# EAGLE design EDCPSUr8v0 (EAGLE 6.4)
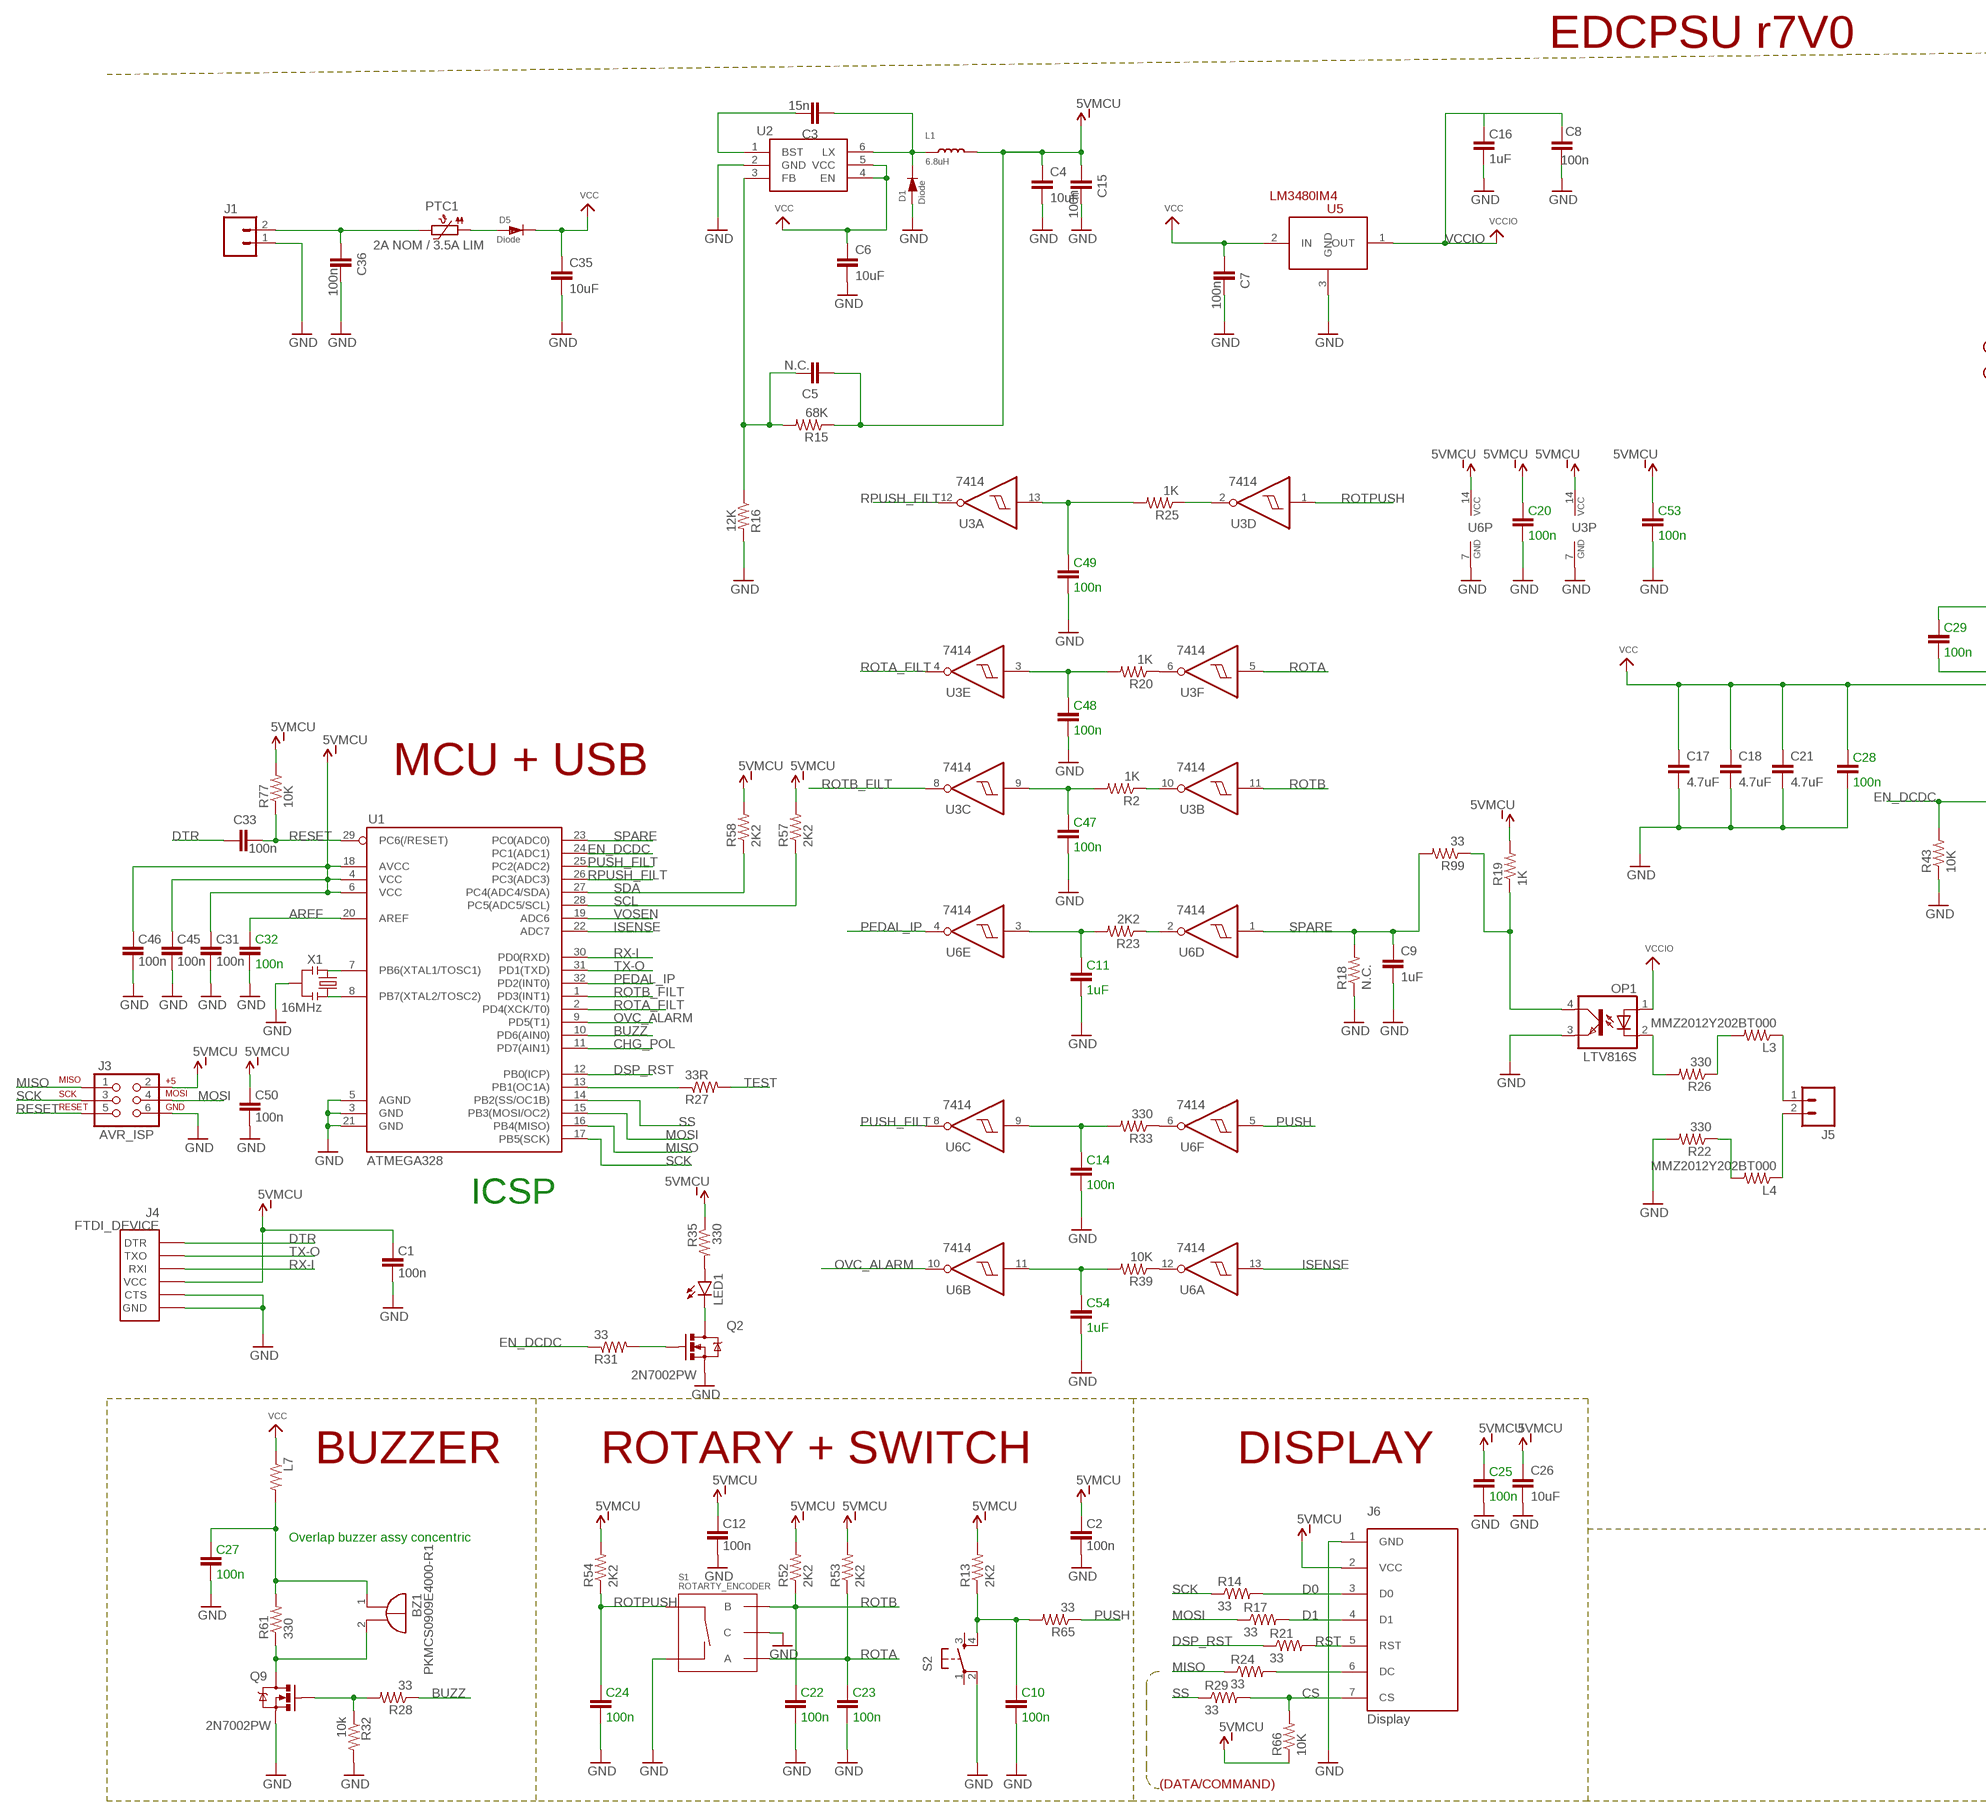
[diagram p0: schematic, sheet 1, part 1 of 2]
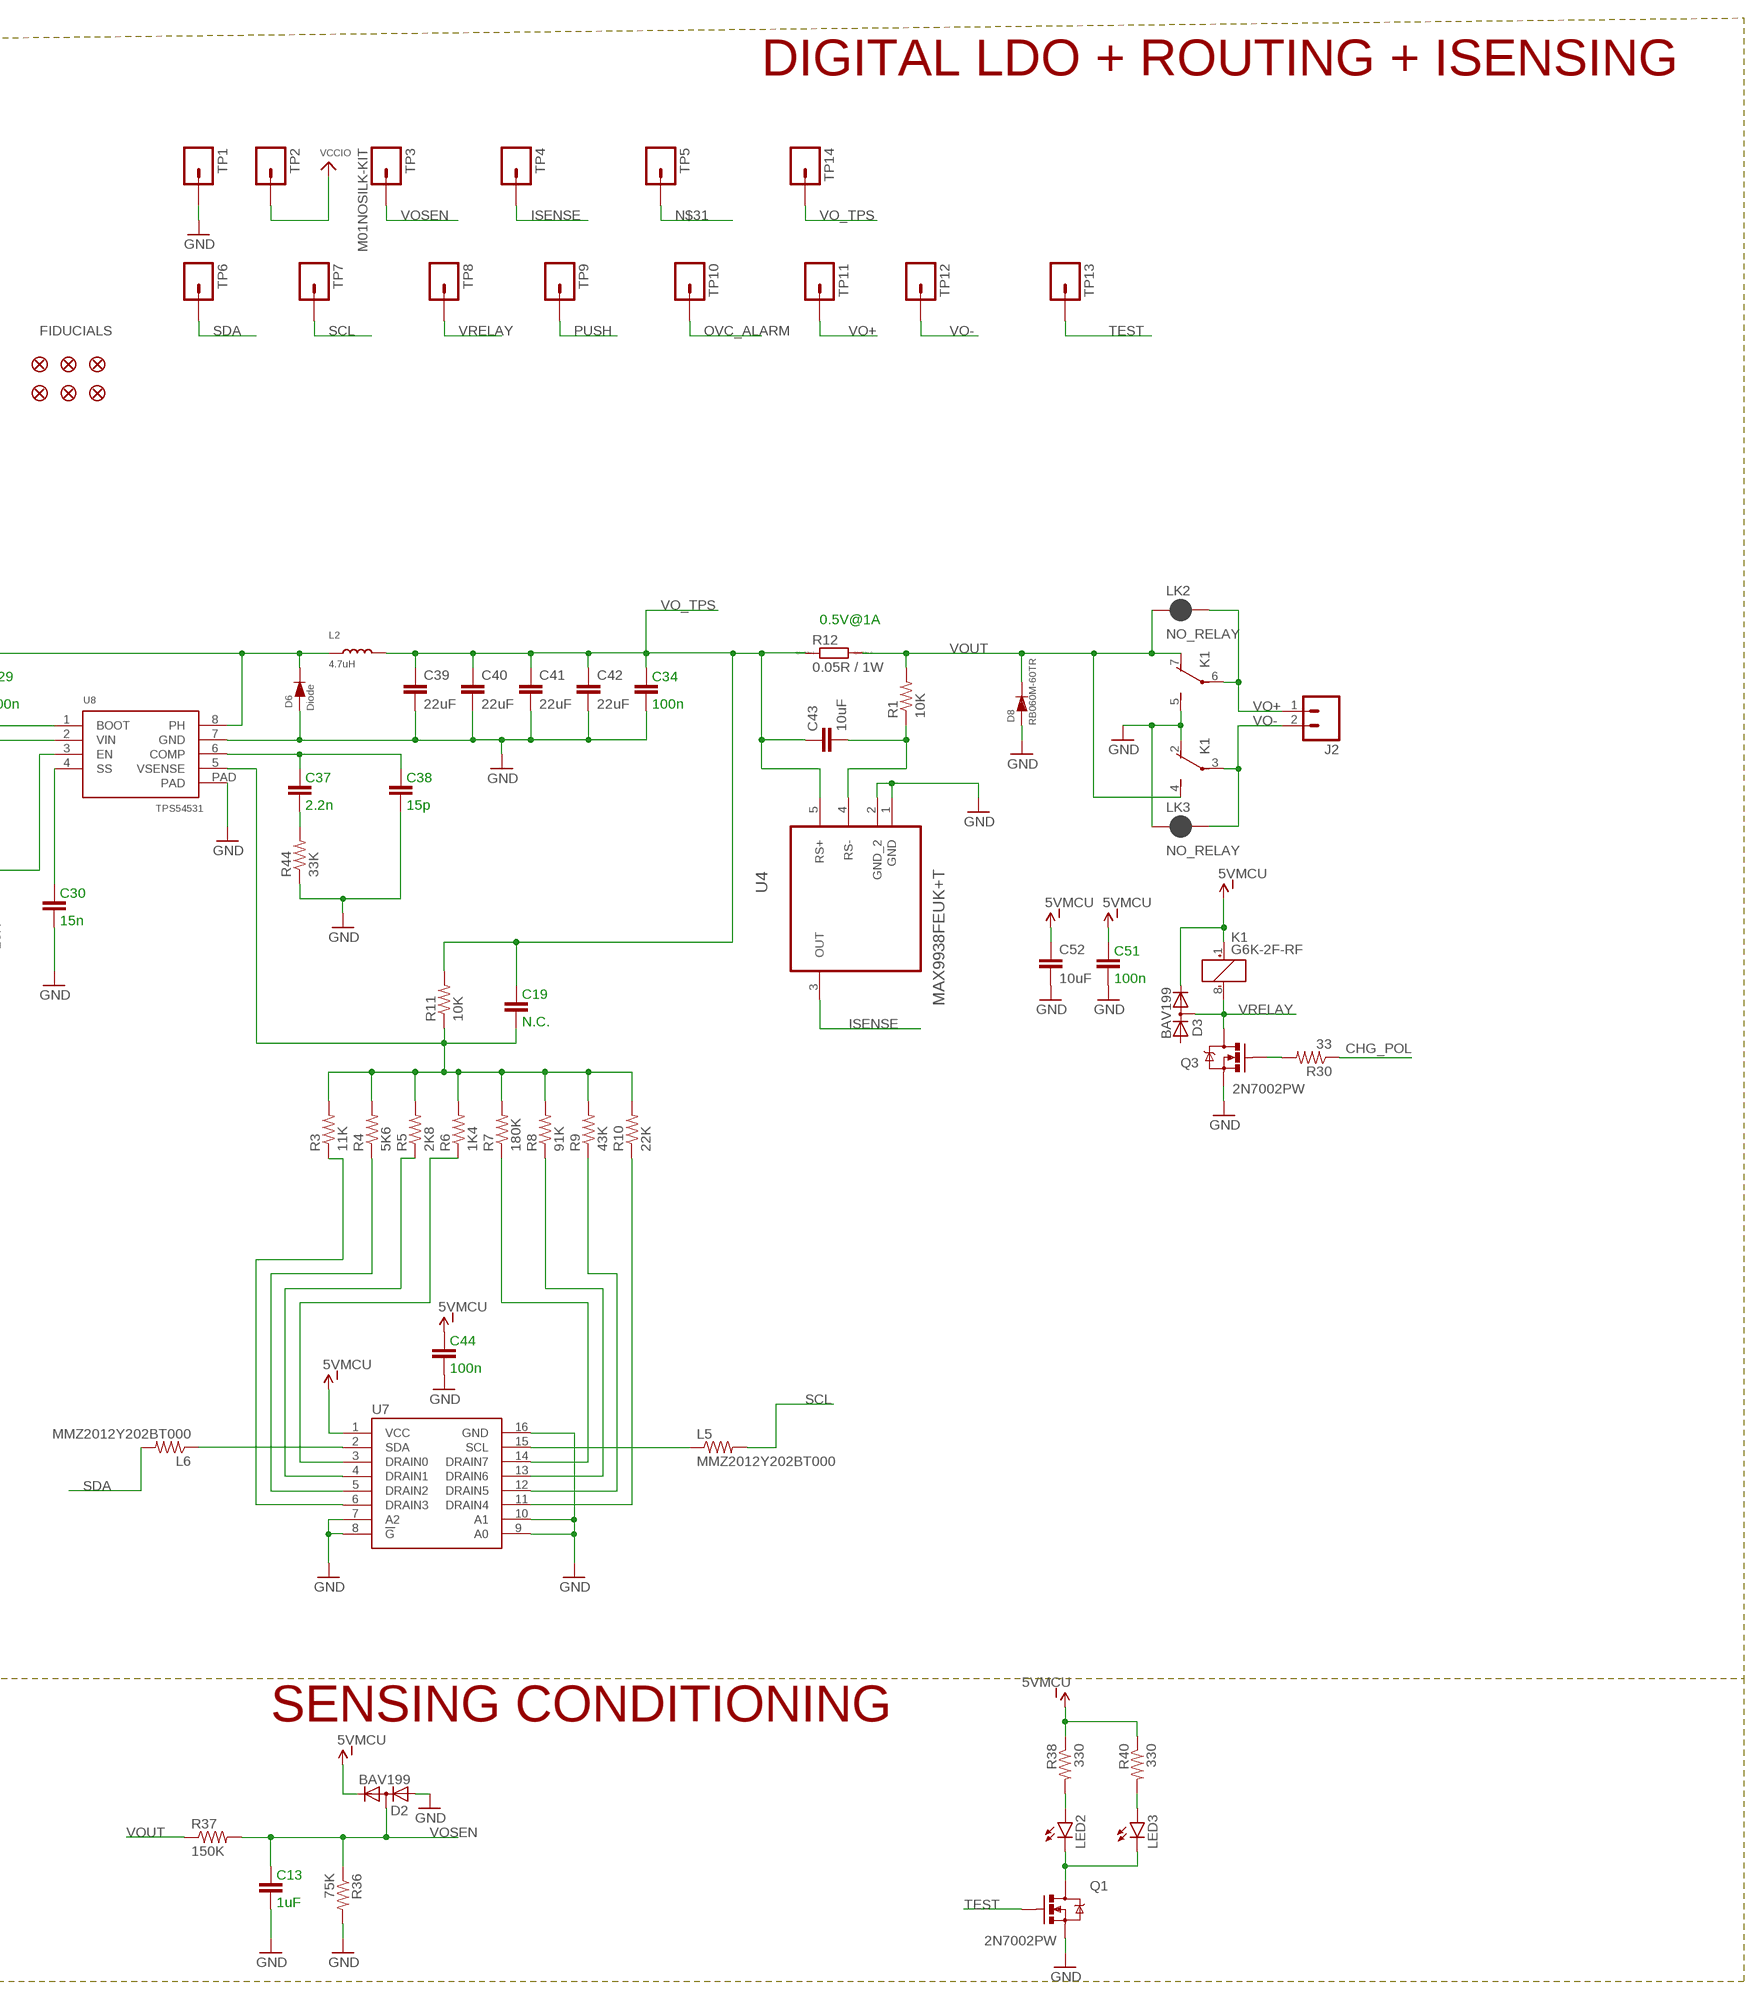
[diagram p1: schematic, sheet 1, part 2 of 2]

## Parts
BZ1  PKMCS0909E4000-R1  [PKMCS0909]
C1  100n  CAP0805  [0805]
C2  100n  CAP0805  [0805]
C3  15n  CAP0805  [0805]
C4  10uF  CAP1206  [1206]
C5  N.C.  CAP0805  [0805]
C6  10uF  CAP1206  [1206]
C7  100n  CAP0805  [0805]
C8  100n  CAP0805  [0805]
C9  1uF  CAP1206  [1206]
C10  100n  CAP0805  [0805]
C11  1uF  CAP0805  [0805]
C12  100n  CAP0805  [0805]
C13  1uF  CAP0805  [0805]
C14  100n  CAP0805  [0805]
C15  100n  CAP0805  [0805]
C16  1uF  CAP0805  [0805]
C17  4.7uF  CAP1210  [1210]
C18  4.7uF  CAP1210  [1210]
C19  N.C.  CAP0805  [0805]
C20  100n  CAP0805  [0805]
C21  4.7uF  CAP1210  [1210]
C22  100n  CAP0805  [0805]
C23  100n  CAP0805  [0805]
C24  100n  CAP0805  [0805]
C25  100n  CAP0805  [0805]
C26  10uF  CAP1206  [1206]
C27  100n  CAP0805  [0805]
C28  100n  CAP0805  [0805]
C29  100n  CAP0805  [0805]
C30  15n  CAP0805  [0805]
C31  100n  CAP0805  [0805]
C32  100n  CAP0805  [0805]
C33  100n  CAP0805  [0805]
C34  100n  CAP0805  [0805]
C35  10uF  CAP1206  [1206]
C36  100n  CAP0805  [0805]
C37  2.2n  CAP0805  [0805]
C38  15p  CAP0805  [0805]
C39  22uF  CAP1210  [1210]
C40  22uF  CAP1210  [1210]
C41  22uF  CAP1210  [1210]
C42  22uF  CAP1210  [1210]
C43  10uF  CAP1206  [1206]
C44  100n  CAP0805  [0805]
C45  100n  CAP0805  [0805]
C46  100n  CAP0805  [0805]
C47  100n  CAP0805  [0805]
C48  100n  CAP0805  [0805]
C49  100n  CAP0805  [0805]
C50  100n  CAP0805  [0805]
C51  100n  CAP0805  [0805]
C52  10uF  CAP1206  [1206]
C53  100n  CAP0805  [0805]
C54  1uF  CAP0805  [0805]
D1  Diode  DSOD123  [SOD123]
D2  BAV199  [SOT23]
D3  BAV199  [SOT23]
D5  Diode  DSMC  [DO-214AB]
D6  Diode  DSMC  [DO-214AB]
D8  RB060M-60TR  DSMA  [SMADIODE]
FID1  FIDUCIAL1X2  [FIDUCIAL-1X2]
FID2  FIDUCIAL1X2  [FIDUCIAL-1X2]
FID3  FIDUCIAL1X2  [FIDUCIAL-1X2]
FID4  FIDUCIAL1X2  [FIDUCIAL-1X2]
FID5  FIDUCIAL1X2  [FIDUCIAL-1X2]
FID6  FIDUCIAL1X2  [FIDUCIAL-1X2]
J1  M02LOCK_LONGPADS  [1X02_LOCK_LONGPADS]
J2  M02LOCK_LONGPADS  [1X02_LOCK_LONGPADS]
J3  AVR_ISP  AVR_SPI_PRG_62X3_LOCK  [2X3_LOCK]
J4  FTDI_DEVICE  [FTDI_DEVICE_SIDE]
J5  M02LOCK_LONGPADS  [1X02_LOCK_LONGPADS]
J6  Display  OLED_LCD  [OLED_LCD]
K1  G6K-2F-RF  [G6K-RF]
L1  6.8uH  L4018  [NR4018T100M]
L2  4.7uH  L74437368047  [WE-LHMI]
L3  MMZ2012Y202BT000  RESISTOR0805-RES  [0805]
L4  MMZ2012Y202BT000  RESISTOR0805-RES  [0805]
L5  MMZ2012Y202BT000  RESISTOR0805-RES  [0805]
L6  MMZ2012Y202BT000  RESISTOR0805-RES  [0805]
L7  MMZ2012Y202BT000  RESISTOR0805-RES  [0805]
LED1  LED3MM  [LED3MM]
LED2  LED5MM  [LED5MM]
LED3  LED5MM  [LED5MM]
LK2  NO_RELAY  JUMPER-PAD-2-NC_BY_PASTE  [PAD-JUMPER-2-NC_BY_PASTE_YES_SILK]
LK3  NO_RELAY  JUMPER-PAD-2-NC_BY_PASTE  [PAD-JUMPER-2-NC_BY_PASTE_YES_SILK]
OP1  LTV816S  [SMD4]
PTC1  2A NOM / 3.5A LIM  PTC-  [1812L]
Q1  2N7002PW  MOSFET-NCHANNEL2N7002PW  [SOT323]
Q2  2N7002PW  MOSFET-NCHANNEL2N7002PW  [SOT323]
Q3  2N7002PW  MOSFET-NCHANNEL2N7002PW  [SOT323]
Q9  2N7002PW  MOSFET-NCHANNEL2N7002PW  [SOT323]
R1  10K  RESISTOR0805-RES  [0805]
R2  1K  RESISTOR0805-RES  [0805]
R3  11K  RESISTOR0805-RES  [0805]
R4  5K6  RESISTOR0805-RES  [0805]
R5  2K8  RESISTOR0805-RES  [0805]
R6  1K4  RESISTOR0805-RES  [0805]
R7  180K  RESISTOR0805-RES  [0805]
R8  91K  RESISTOR0805-RES  [0805]
R9  43K  RESISTOR0805-RES  [0805]
R10  22K  RESISTOR0805-RES  [0805]
R11  10K  RESISTOR0805-RES  [0805]
R12  0.05R / 1W  RR2512  [R2512]
R13  2K2  RESISTOR0805-RES  [0805]
R14  33  RESISTOR0805-RES  [0805]
R15  68K  RESISTOR0805-RES  [0805]
R16  12K  RESISTOR0805-RES  [0805]
R17  33  RESISTOR0805-RES  [0805]
R18  N.C.  RESISTOR0805-RES  [0805]
R19  1K  RESISTOR0805-RES  [0805]
R20  1K  RESISTOR0805-RES  [0805]
R21  33  RESISTOR0805-RES  [0805]
R22  330  RESISTOR1206  [1206]
R23  2K2  RESISTOR0805-RES  [0805]
R24  33  RESISTOR0805-RES  [0805]
R25  1K  RESISTOR0805-RES  [0805]
R26  330  RESISTOR1206  [1206]
R27  33R  RESISTOR0805-RES  [0805]
R28  33  RESISTOR0805-RES  [0805]
R29  33  RESISTOR0805-RES  [0805]
R30  33  RESISTOR0805-RES  [0805]
R31  33  RESISTOR0805-RES  [0805]
R32  10k  RESISTOR0805-RES  [0805]
R33  330  RESISTOR0805-RES  [0805]
R35  330  RESISTOR0805-RES  [0805]
R36  75K  RESISTOR0805-RES  [0805]
R37  150K  RESISTOR0805-RES  [0805]
R38  330  RESISTOR0805-RES  [0805]
R39  10K  RESISTOR0805-RES  [0805]
R40  330  RESISTOR0805-RES  [0805]
R43  10K  RESISTOR0805-RES  [0805]
R44  33K  RESISTOR0805-RES  [0805]
R52  2K2  RESISTOR0805-RES  [0805]
R53  2K2  RESISTOR0805-RES  [0805]
R54  2K2  RESISTOR0805-RES  [0805]
R57  2K2  RESISTOR0805-RES  [0805]
R58  2K2  RESISTOR0805-RES  [0805]
R61  330  RESISTOR0805-RES  [0805]
R65  33  RESISTOR0805-RES  [0805]
R66  10K  RESISTOR0805-RES  [0805]
R77  10K  RESISTOR0805-RES  [0805]
R99  33  RESISTOR0805-RES  [0805]
S1  ROTARTY_ENCODER  [ROTARY_ENC_PLAIN]
S2  TAC_SWITCH_KSC931G-SMD  [TAC_SW_SMD_KSC931G]
TP1  M01POGOPIN_HOLE_LARGE  [1X01_POGOPIN_HOLE_LARGE]
TP2  M01POGOPIN_HOLE_LARGE  [1X01_POGOPIN_HOLE_LARGE]
TP3  M01NOSILK-KIT  [1X01NS-KIT]
TP4  M01POGOPIN_HOLE_LARGE  [1X01_POGOPIN_HOLE_LARGE]
TP5  M01POGOPIN_HOLE_LARGE  [1X01_POGOPIN_HOLE_LARGE]
TP6  M01POGOPIN_HOLE_LARGE  [1X01_POGOPIN_HOLE_LARGE]
TP7  M01POGOPIN_HOLE_LARGE  [1X01_POGOPIN_HOLE_LARGE]
TP8  M01POGOPIN_HOLE_LARGE  [1X01_POGOPIN_HOLE_LARGE]
TP9  M01POGOPIN_HOLE_LARGE  [1X01_POGOPIN_HOLE_LARGE]
TP10  M01POGOPIN_HOLE_LARGE  [1X01_POGOPIN_HOLE_LARGE]
TP11  M01POGOPIN_HOLE_LARGE  [1X01_POGOPIN_HOLE_LARGE]
TP12  M01POGOPIN_HOLE_LARGE  [1X01_POGOPIN_HOLE_LARGE]
TP13  M01POGOPIN_HOLE_LARGE  [1X01_POGOPIN_HOLE_LARGE]
TP14  M01POGOPIN_HOLE_LARGE  [1X01_POGOPIN_HOLE_LARGE]
U1  ATMEGA328  ATMEGA168  [TQFP32-08]
U2  BD9G101G  [SSOP6]
U3  7414  [TSSOP14]
U4  MAX9938FEUK+T  [SOT95P280X145-5N]
U5  LM3480IM4  [SOT23-3]
U6  7414  [TSSOP14]
U7  TPIC2810D  [SO16]
U8  TPS54531  TPS5431DDAR  [SOIC8]
X1  16MHz  RESONATORSMD  [RESONATOR-SMD]

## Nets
AREF: C32.2 U1.20(AREF)
BUZZ: R28.1 U1.10(PD6(AIN0))
CHG_POL: R30.1 U1.11(PD7(AIN1))
CS: J6.7(CS) R29.2 R66.2
D0: J6.3(D0) R14.2
D1: J6.4(D1) R17.2
DSP_RST: R21.1 U1.12(PB0(ICP))
DTR: C33.2 J4.P$1(DTR)
EN_DCDC: R31.1 R43.2 U1.24(PC1(ADC1)) U8.3(EN)
GND: C1.1 C2.1 C4.2 C6.2 C7.1 C8.1 C9.2 C10.1 C11.1 C12.1 C13.1 C14.1 C15.1 C16.1 C17.2 C18.2 C20.1 C21.2 C22.1 C23.1 C24.1 C25.1 C26.2 C27.1 C28.1 C30.1 C31.1 C32.1 C34.1 C35.2 C36.1 C38.1 C39.2 C40.2 C41.2 C42.2 C44.1 C45.1 C46.1 C47.1 C48.1 C49.1 C50.1 C51.1 C52.2 C53.1 C54.1 D1.+(A) D2.1(A) D6.1(A) D8.A J1.1 J3.6 J4.P$5(CTS) J4.P$6(GND) J6.1(GND) K1.2(A:O) K1.5(B:S) LK3.1 OP1.3(EMIT) Q1.2(S) Q2.2(S) Q3.2(S) Q9.2(S) R16.2 R18.1 R22.2 R32.2 R36.2 R43.1 R44.1 S1.C S1.SW- S2.2 TP1.1 U1.3(GND) U1.5(AGND) U1.21(GND) U2.2(GND) U3.7(P:GND) U4.1(GND) U4.2(GND_2) U5.3(GND) U6.7(P:GND) U7.7(A2) U7.8(!G) U7.9(A0) U7.10(A1) U7.16(GND) U8.7(GND) U8.PAD X1.2
ISENSE: TP4.1 U1.22(ADC7) U4.3(OUT) U6.13(A:I)
MISO: J3.1 R24.1 U1.16(PB4(MISO))
MOSI: J3.4 R17.1 U1.15(PB3(MOSI/OC2))
N$1: R3.1 U7.6(DRAIN3)
N$2: R4.1 U7.5(DRAIN2)
N$3: R5.1 U7.4(DRAIN1)
N$4: R6.1 U7.3(DRAIN0)
N$5: R7.1 U7.14(DRAIN7)
N$6: J6.6(DC) R24.2
N$7: R8.1 U7.13(DRAIN6)
N$8: R9.1 U7.12(DRAIN5)
N$9: R10.1 U7.11(DRAIN4)
N$10: C43.2 R1.1 U4.4(RS-)
N$11: LED1.A R35.2
N$12: LED1.K(C) Q2.3(D)
N$13: R33.1 U6.6(F:O)
N$14: D5.1(A) PTC1.1
N$15: R39.1 U6.12(A:O)
N$16: C3.1 U2.1(BST)
N$17: C10.2 R13.1 R65.2 S2.4
N$18: C47.2 R2.2 U3.9(C:I)
N$19: C3.2 D1.-(K) L1.1 U2.6(LX)
N$20: Q9.1(G) R28.2 R32.1
N$21: Q2.1(G) R31.2
N$22: R2.1 U3.10(B:O)
N$23: R20.1 U3.6(F:O)
N$24: U1.8(PB7(XTAL2/TOSC2)) X1.1
N$25: R25.1 U3.2(D:O)
N$26: C49.2 R25.2 U3.13(A:I)
N$27: C5.1 R15.2 R16.1 U2.3(FB)
N$28: C48.2 R20.2 U3.3(E:I)
N$29: C11.2 R23.2 U6.3(E:I)
N$30: R27.1 U1.13(PB1(OC1A))
N$31: OP1.4(COL) R19.1 R99.1 TP5.1
N$32: BZ1.1(+) C27.2 L7.2 R61.2
N$33: C36.2 J1.2 PTC1.2
N$34: R23.1 U6.2(D:O)
N$36: U1.7(PB6(XTAL1/TOSC1)) X1.3
N$37: C14.2 R33.2 U6.9(C:I)
N$38: LED2.A R38.2
N$39: C54.2 R39.2 U6.11(B:I)
N$40: L6.1 U7.2(SDA)
N$41: OP1.2(C) R26.2
N$42: Q3.1(G) R30.2
N$43: L3.2 R26.1
N$44: C30.2 U8.4(SS)
N$46: L4.2 R22.1
N$47: C29.1 U8.1(BOOT)
N$48: C19.1 R3.2 R4.2 R5.2 R6.2 R7.2 R8.2 R9.2 R10.2 R11.1 U8.5(VSENSE)
N$49: LED3.A R40.2
N$51: C29.2 D6.2(K) L2.1 U8.8(PH)
N$52: C37.2 C38.2 U8.6(COMP)
N$53: C37.1 R44.2
N$54: L5.1 U7.15(SCL)
N$55: J5.1 L3.1
N$56: J5.2 L4.1
N$57: LED2.K(C) LED3.K(C) Q1.3(D)
N$64: BZ1.2(-) Q9.3(D) R61.1
OVC_ALARM: TP10.1 U1.9(PD5(T1)) U6.10(B:O)
PEDAL_IP: U1.32(PD2(INT0)) U6.4(E:O)
PUSH: R65.1 TP9.1 U6.5(F:I)
PUSH_FILT: U1.25(PC2(ADC2)) U6.8(C:O)
RESET: C33.1 J3.5 R77.1 U1.29(PC6(/RESET))
ROTA: C23.2 R53.1 S1.A U3.5(F:I)
ROTA_FILT: U1.2(PD4(XCK/T0)) U3.4(E:O)
ROTB: C22.2 R52.1 S1.B U3.11(B:I)
ROTB_FILT: U1.1(PD3(INT1)) U3.8(C:O)
ROTPUSH: C24.2 R54.1 S1.SW+ U3.1(D:I)
RPUSH_FILT: U1.26(PC3(ADC3)) U3.12(A:O)
RST: J6.5(RST) R21.2
RX-I: J4.P$3(RXI) U1.30(PD0(RXD))
SCK: J3.3 R14.1 U1.17(PB5(SCK))
SCL: L5.2 R57.1 TP7.1 U1.28(PC5(ADC5/SCL))
SDA: L6.2 R58.1 TP6.1 U1.27(PC4(ADC4/SDA))
SPARE: C9.1 R18.2 R99.2 U1.23(PC0(ADC0)) U6.1(D:I)
SS: R29.1 U1.14(PB2(SS/OC1B))
TEST: Q1.1(G) R27.2 TP13.1
TX-O: J4.P$2(TXO) U1.31(PD1(TXD))
VCC: C6.1 C7.2 C17.1 C18.1 C21.1 C28.2 C35.1 D5.2(K) L7.1 U2.4(EN) U2.5(VCC) U5.2(IN) U8.2(VIN)
VCC-ISO: C1.2 C2.2 C4.1 C5.2 C12.2 C15.2 C20.2 C25.2 C26.1 C31.2 C44.2 C45.2 C46.2 C50.2 C51.2 C52.1 C53.2 D2.2(C) D3.2(C) J3.2 J4.P$4(VCC) J6.2(VCC) K1.1(1:+) L1.2 R13.2 R15.1 R19.2 R35.1 R38.1 R40.1 R52.2 R53.2 R54.2 R57.2 R58.2 R66.1 R77.2 U1.4(VCC) U1.6(VCC) U1.18(AVCC) U3.14(P:VCC) U6.14(P:VCC) U7.1(VCC) ; supply symbol labelled 5VMCU
VCCIO: C8.2 C16.2 OP1.1(A) TP2.1 U5.1(OUT)
VO+: J2.1 K1.6(B:P) LK2.2 TP11.1
VO-: J2.2 K1.3(A:P) LK3.2 TP12.1
VO_TPS: C19.2 C34.2 C39.1 C40.1 C41.1 C42.1 C43.1 L2.2 R11.2 R12.1 TP14.1 U4.5(RS+)
VOSEN: C13.2 D2.3(AC) R36.1 R37.2 TP3.1 U1.19(ADC6)
VOUT: D8.C(K) K1.4(A:S) K1.7(B:O) LK2.1 R1.2 R12.2 R37.1
VRELAY: D3.3(AC) K1.8(1:-) Q3.3(D) TP8.1
Unconnected: D3.1(A) K1.A(S1:SH) K1.B(S2:SH) S2.1 S2.3

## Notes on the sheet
- EDCPSU r7V0
- DIGITAL LDO + ROUTING + ISENSING
- FIDUCIALS
- 0.5V@1A
- MCU + USB
- ICSP
- BUZZER | ROTARY + SWITCH | DISPLAY
- Overlap buzzer assy concentric
- SENSING CONDITIONING
- (DATA/COMMAND)

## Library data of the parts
BZ1 = buzzer:PKMCS0909E4000-R1: PKMCS0909E4000-R1
C1-C3 C5 C7 C8 C10-C16 C19 C20 C22-C25 C27-C34 C36-C38 C44-C51 C53 C54 = SparkFun:CAP: Capacitor
C4 C6 C9 C17 C18 C21 C26 C35 C39-C43 C52 = SparkFun-Passives:CAP: Capacitor
D1 D5 D6 D8 = EDCPSU - Rev3:D*
D2 D3 = diode:BAV199: DIODE low-leakage double diode
FID1-FID6 = SparkFun-Aesthetics:FIDUCIAL: Fiducial Alignment Points
J1 J2 J5 = SparkFun-Connectors:M02: Standard 2-pin 0.1" header. Use with
J3 = SparkFun-Connectors:AVR_SPI_PRG_6: AVR ISP 6 Pin This is the reduced ISP connector for AVR programming. Common on Arduino. This footprint will take up less PCB space and can be used with a 10-pin to 6-pin adapter such as SKU: BOB-08508 **Special note about "TEST_POINT" package. The stop mask is on the top side, so if you want your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
J4 = SparkFun-Connectors:FTDI_DEVICE: Connector which mates to FTDI basic or FTDI cable.
J6 = EDCPSU:OLED_LCD
K1 = relay:G6K*-2F-RF: OMRON High Frequency Relay G6K-RF Compact High Frequency Relays with 2 Form C (DPDT) Contacts Handles 1 A, 30 VDC discrete load and 1 W at 1 GHz high frequency load D20G6KRF0602.pdf; MF: OMRON COMPONENTS USA; MPN: G6K-2F-RF-DC12; OC_FARNELL: 1448181; OC_NEWARK: 73C8948
L1 L2 = EDCPSU - Rev3:L*
L3-L7 R1-R11 R13-R21 R23-R25 R27-R33 R35-R40 R43 R44 R52-R54 R57 R58 R61 R65 R66 R77 R99 = SparkFun:RESISTOR: Resistor
LED1-LED3 = SparkFun-LED:LED: LEDs
LK2 LK3 = SparkFun-Passives:JUMPER-PAD-2-NC_BY_PASTE
OP1 = optocoupler:LTV816: OPTO COUPLER Source: LITEON, LTV816.pdf; OC_FARNELL: unknown; OC_NEWARK: unknown
PTC1 = EDCPSU:PTC-: Positive Temperature Coefficient Resistor (PTC)
Q1-Q3 Q9 = SparkFun-DiscreteSemi:MOSFET-NCHANNEL: Common NMOSFET Parts MFG P/NStore IDProd ID FDD8780TRANS-09984 SI7820DNTRANS-11055 FDS6630AIC-08089 2N7002PWTRANS-11151 FQP30N06L COM-10213TRANS-10060 BSS123LT1GTRANS-08345 BSS138TRANS-00830 BS170 2N7000; PROD_ID: TRANS-11151
R12 = eagle-ltspice:R: RESISTOR, European symbol; SPICEMODEL: NONE; SPICEPREFIX: R
R22 R26 = SparkFun-Passives:RESISTOR: Resistor
S1 = SparkFun-Electromechanical:ROTARTY_ENCODER: Simple no LED rotary encoder Example: COM-09117
S2 = EDCPSU - Rev2:TAC_SWITCH: Momentary Switch Button commonly used for reset or general input. Spark Fun Electronics SKU : COM-00097 SMT- SWCH-08247
TP1-TP14 = SparkFun-Connectors:M01: Header 1
U1 = SparkFun:ATMEGA168
U2 = EDCPSU - Rev3:BD9G101G: BD9G101G - Simple Step-down Switching Regulators with Built-in Power MOSFET
U3 U6 = 74xx-eu:74*14: Hex schmitt trigger INVERTER
U4 = MAX9938:MAX9938FEUK+T; DESCRIPTION: Precision Current-Sense Amplifier; MPN: MAX9938FEUK+T; OC_FARNELL: -; OC_NEWARK: 01N6733; PACKAGE: SOT-23-5; SUPPLIER: Maxim
U5 = SparkFun-PowerIC:LM3480IM4: Small package linear regulator
U7 = EDCPSU - Rev2:TPIC2810D
U8 = EDCPSU - Rev3:TPS5431DDAR: Source : http://www.ti.com/lit/ds/symlink/tps54531.pdf
X1 = SparkFun:RESONATOR: Resonator Small SMD resonator. This is the itty bitty 10/20MHz resonators with built in caps. CSTCE10M0G55 and CSTCE20M0V53. Footprint has been reviewed closely but hasn't been tested yet.

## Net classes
1 vcc: width 0.254 mm

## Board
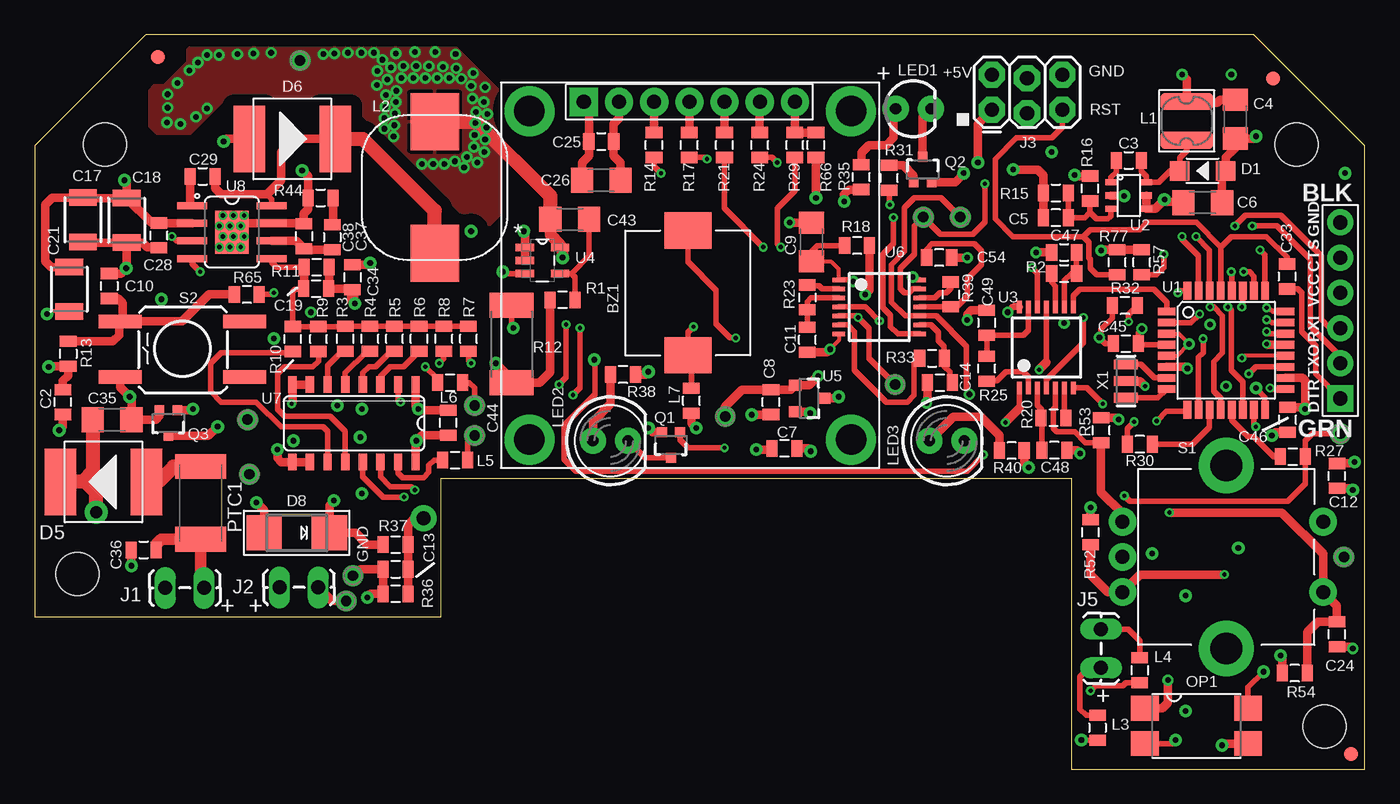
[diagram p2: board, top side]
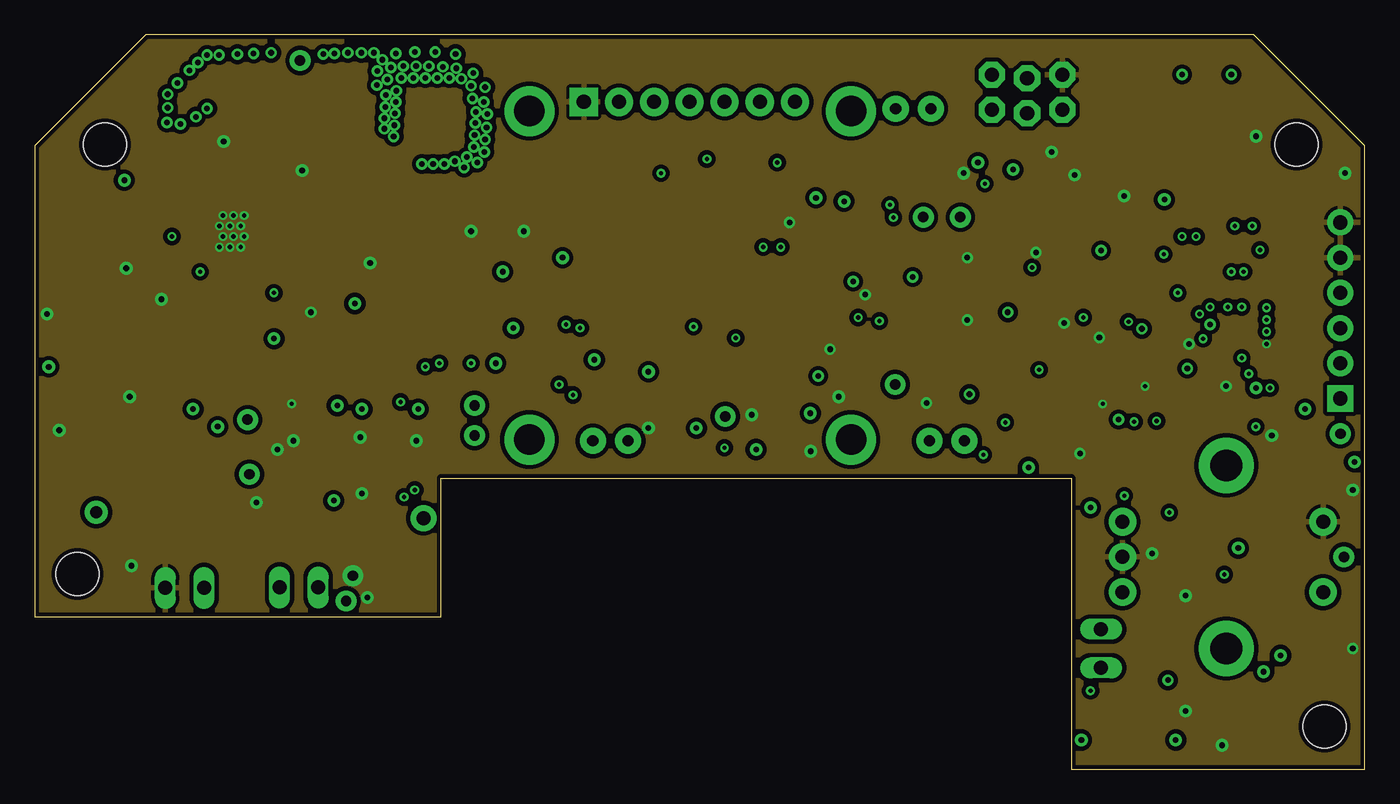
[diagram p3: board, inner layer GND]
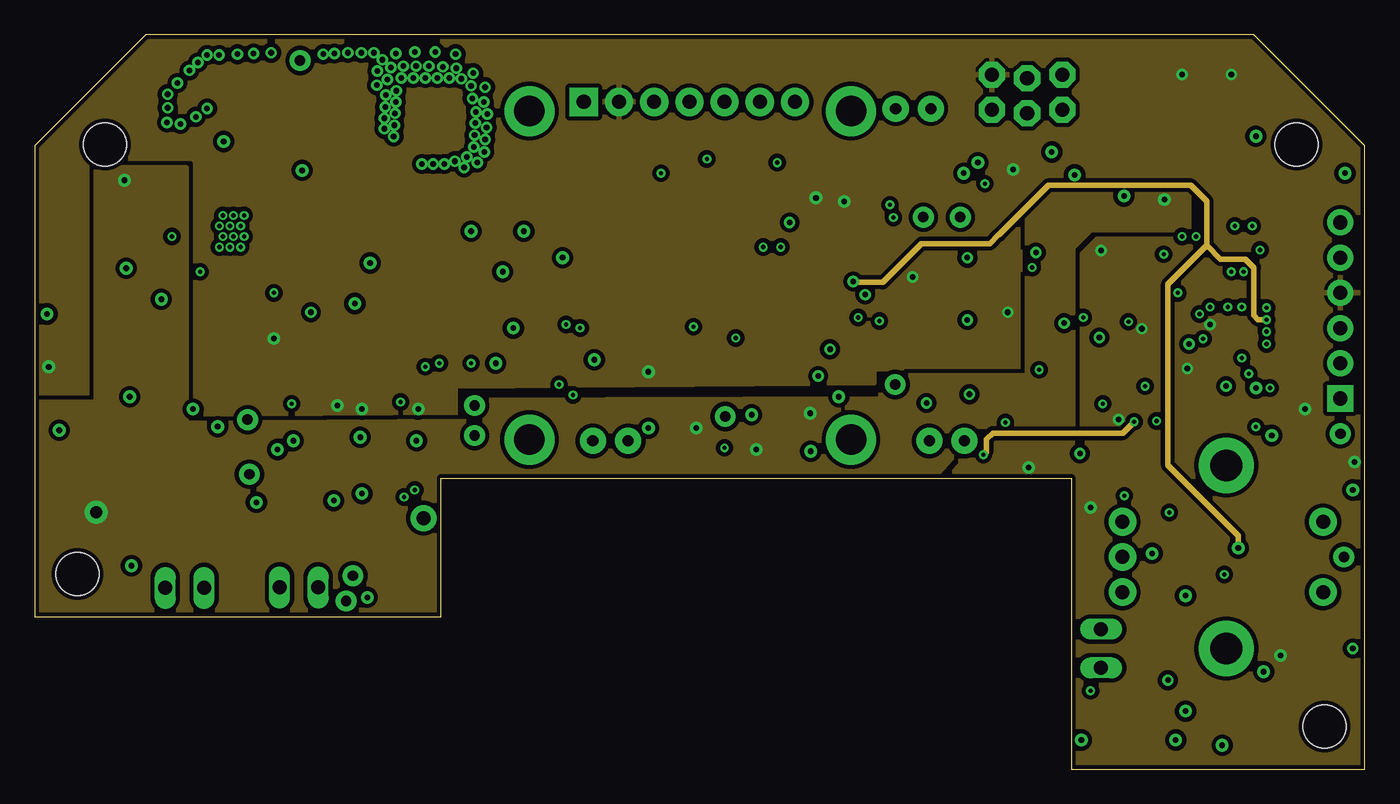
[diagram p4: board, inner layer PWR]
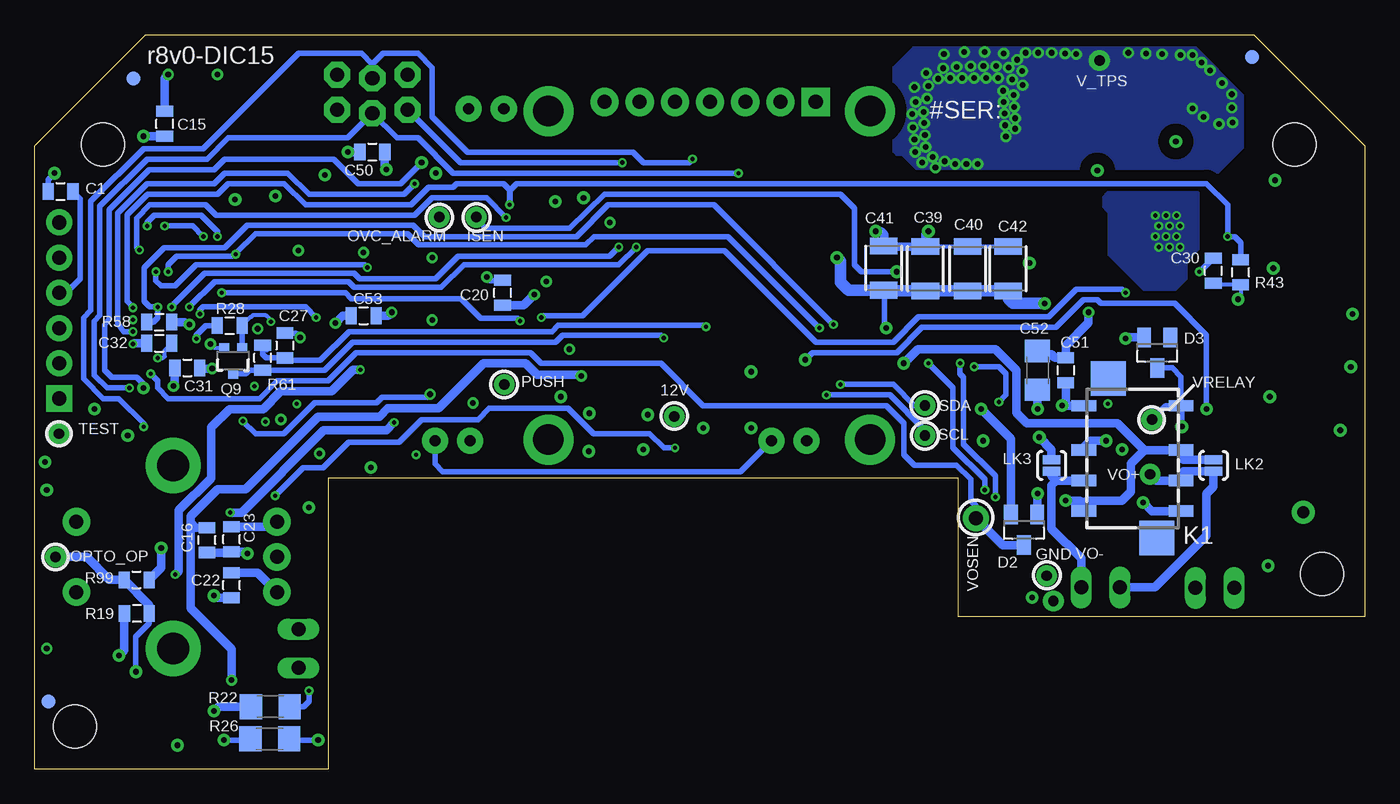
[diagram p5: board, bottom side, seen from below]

Size 96 x 53 mm. Coordinates in mm from the lower left corner, seen from the top.
Outline: 96,0 96,45 88,53 8,53 0,45 0,11 29.35,11 29.35,21 74.81,21 74.81,0 96,0
Copper layers (1*2*15*16): Top 0.035mm / dielectric 1.5mm / GND 0.0175mm / dielectric 1.1mm / PWR 0.0175mm / dielectric 0.2mm / Bottom 0.035mm
Design rules "SeeedStudio_2layer_DRU_no_angle_20140221 *": minimum track width 6mil, minimum drill 12mil, track to track 6mil, track to pad 6mil, pad to pad 6mil, via to via 6mil, smd to smd 0mil, copper to edge 10mil, drill to drill 10mil, minimum pad ring 10mil, minimum via ring 6mil, stop-mask expansion 2mil, vias tented up to drill 100mil, thermal gap 10mil
Holes 3.1 mm at 5.08,45.08 91.08,45.08 3.08,14.08 93.08,3.08

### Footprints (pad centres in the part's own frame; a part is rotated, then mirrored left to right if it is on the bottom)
PKMCS0909 = smd 2.6 x 3.4: 1 -4.5,0; 2 4.5,0
0805 = smd 0.8 x 1.2: 1 -0.9,0; 2 0.9,0
1206 = smd 1.6 x 1.8: 1 -1.4,0; 2 1.4,0
1210 = smd 1.2 x 2: 1 -1.6,0; 2 1.6,0
SOD123 = smd 1.397 x 1.397: + -1.651,0; - 1.651,0
SOT23 = smd 1 x 1.4: 1 -0.95,-1.1; 2 0.95,-1.1; 3 0,1.1
DO-214AB = smd 2.286 x 4.8: 1 -3.1,0; 2 3.1,0
SMADIODE = smd 2.54 x 2.54: A 2.349,0; C -2.349,0
FIDUCIAL-1X2 = smd 1 x 1: 1 0,0
1X02_LOCK_LONGPADS = drill 1.016 long: 1 -0.127,0; 2 2.667,0
2X3_LOCK = drill 1.016 pad 1.88 octagon: 1 0,0; 2 0,2.54; 3 2.54,-0.254; 4 2.54,2.286; 5 5.08,0; 6 5.08,2.54
FTDI_DEVICE_SIDE = drill 1.016 pad 1.88 square: P$1 -6.35,0 | drill 1.016 pad 1.88: P$2 -3.81,0; P$3 -1.27,0; P$4 1.27,0; P$5 3.81,0; P$6 6.35,0
OLED_LCD = drill 1.016 pad 2.032 square: 1 -7.42,13.7 | drill 1.016 pad 2.032: 2 -4.88,13.7; 3 -2.34,13.7; 4 0.2,13.7; 5 2.74,13.7; 6 5.28,13.7; 7 7.82,13.7 | drill 2.2 pad 3.6: M1 -11.34,13.04; M2 11.86,13.04; M3 11.86,-10.66; M4 -11.34,-10.66
G6K-RF = smd 0.8 x 1.8: 1 -3.8,-3.5; 2 -0.6,-3.5; 3 1.6,-3.5; 4 3.8,-3.5; 5 3.8,3.5; 6 1.6,3.5; 7 -0.6,3.5; 8 -3.8,3.5 | smd 2.5 x 2.5: A -5.75,-1.75; B 5.75,1.75
NR4018T100M = smd 1.25 x 3.8: 1 -1.4,0; 2 1.4,0
WE-LHMI = smd 4.1 x 3.5: 1 -4.75,0; 2 4.75,0
LED3MM = drill 0.813 pad 1.88: A -1.27,0; K 1.27,0
LED5MM = drill 0.813 pad 1.88: A -1.27,0; K 1.27,0
PAD-JUMPER-2-NC_BY_PASTE_YES_SILK = smd 0.635 x 1.27: 1 -0.401,0; 2 0.413,0
SMD4 = smd 1.78 x 2: 1 -1.27,-3.725; 2 1.27,-3.725; 3 1.27,3.725; 4 -1.27,3.725
1812L = smd 1.8 x 3.7: 1 -2.6,0; 2 2.65,0
SOT323 = smd 0.7 x 0.7: 1 -0.65,-0.925; 2 0.65,-0.925; 3 0,0.925
R2512 = smd 1.8 x 3.2: 1 -2.8,0; 2 2.8,0
ROTARY_ENC_PLAIN = drill 1.016 pad 2: A 7.493,-2.54; B 7.493,2.54; C 7.493,0; SW+ -6.985,2.54; SW- -6.985,-2.54 | drill 2.286 pad 4: P$3 0,6.604; P$4 0,-6.604
TAC_SW_SMD_KSC931G = smd 3.1 x 1: 1 -4.5,2; 2 4.5,2; 3 -4.5,-2; 4 4.5,-2
1X01_POGOPIN_HOLE_LARGE = drill 0.75 pad 1.5: 1 0,0
1X01NS-KIT = drill 1.016 pad 1.88: 1 0,0
TQFP32-08 = smd 1.27 x 0.559: 1 -4.293,2.8; 2 -4.293,2; 3 -4.293,1.2; 4 -4.293,0.4; 5 -4.293,-0.4; 6 -4.293,-1.2; 7 -4.293,-2; 8 -4.293,-2.8; 17 4.293,-2.8; 18 4.293,-2; 19 4.293,-1.2; 20 4.293,-0.4; 21 4.293,0.4; 22 4.293,1.2; 23 4.293,2; 24 4.293,2.8 | smd 0.559 x 1.27: 9 -2.8,-4.293; 10 -2,-4.293; 11 -1.2,-4.293; 12 -0.4,-4.293; 13 0.4,-4.293; 14 1.2,-4.293; 15 2,-4.293; 16 2.8,-4.293; 25 2.8,4.293; 26 2,4.293; 27 1.2,4.293; 28 0.4,4.293; 29 -0.4,4.293; 30 -1.2,4.293; 31 -2,4.293; 32 -2.8,4.293
SSOP6 = smd 0.8 x 0.45: 1 -1.275,0.95; 2 -1.275,0; 3 -1.275,-0.95; 4 1.275,-0.95; 5 1.275,0; 6 1.275,0.95
TSSOP14 = smd 0.35 x 0.9: 1 -1.95,-2.925; 2 -1.3,-2.925; 3 -0.65,-2.925; 4 0,-2.925; 5 0.65,-2.925; 6 1.3,-2.925; 7 1.95,-2.925; 8 1.95,2.925; 9 1.3,2.925; 10 0.65,2.925; 11 0,2.925; 12 -0.65,2.925; 13 -1.3,2.925; 14 -1.95,2.925
SOT95P280X145-5N = smd 1.321 x 0.559: 1 -1.27,0.94; 2 -1.27,0; 3 -1.27,-0.94; 4 1.27,-0.94; 5 1.27,0.94
SOT23-3 = smd 0.8 x 0.9: 1 -0.95,-1; 2 0.95,-1; 3 0,1.1
SO16 = smd 0.6 x 1.2: 1 -4.445,-2.8; 2 -3.175,-2.8; 3 -1.905,-2.8; 4 -0.635,-2.8; 5 0.635,-2.8; 6 1.905,-2.8; 7 3.175,-2.8; 8 4.445,-2.8; 9 4.445,2.8; 10 3.175,2.8; 11 1.905,2.8; 12 0.635,2.8; 13 -0.635,2.8; 14 -1.905,2.8; 15 -3.175,2.8; 16 -4.445,2.8
SOIC8 = smd 2.15 x 0.5: 1 -2.875,1.905; 2 -2.875,0.635; 3 -2.875,-0.635; 4 -2.875,-1.905; 5 2.875,-1.905; 6 2.875,-0.635; 7 2.875,0.635; 8 2.875,1.905 | smd 2.4 x 3.1: PAD 0,0
RESONATOR-SMD = smd 0.7 x 1.7: 1 -1.2,0; 2 0,0; 3 1.2,0

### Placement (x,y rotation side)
BZ1  47.14,34.37 90 top
C1  94.13,41.68 0 bottom
C2  2.03,26.49 90 top
C3  78.96,43.93 0 top
C4  86.65,46.9 270 top
C5  73.7,39.79 180 top
C6  84.29,40.88 0 top
C7  54.1,23.15 180 top
C8  53.14,26.49 90 top
C9  56.06,38.04 90 top
C10  5.38,34.86 270 top
C11  55.77,30.99 90 top
C12  93.98,21.16 90 top
C13  26.06,14.43 0 top
C14  65.34,27.89 0 top
C15  86.61,46.56 90 bottom
C16  83.57,16.54 90 bottom
C17  3.48,39.65 270 top
C18  6.64,39.6 270 top
C19  20.32,34.67 0 top
C20  62.23,34.37 90 bottom
C21  2.49,34.63 270 top
C22  81.79,13.29 90 bottom
C23  81.79,16.59 90 bottom
C24  93.98,9.73 90 top
C25  40.89,45.29 0 top
C26  40.89,42.5 180 top
C27  77.94,30.57 270 bottom
C28  8.97,38.51 90 top
C29  12.13,42.78 0 top
C30  10.93,35.96 90 bottom
C31  84.98,28.96 0 bottom
C32  87.01,30.74 0 bottom
C33  90.39,35.55 270 top
C34  22.94,35.49 270 top
C35  5.59,25.22 0 top
C36  7.87,15.83 0 top
C37  21.48,38.38 270 top
C38  19.44,38.44 270 top
C39  31.71,36.11 90 bottom
C40  28.66,36.11 90 bottom
C41  34.72,36.16 90 bottom
C42  25.74,36.11 90 bottom
C43  38.62,39.66 0 top
C44  29.84,25.01 90 top
C45  78.74,30.71 0 top
C46  90.42,25.22 90 top
C47  74.3,37.29 0 top
C48  73.58,23.01 180 top
C49  68.71,32.21 270 top
C50  71.63,44.53 0 bottom
C51  21.59,28.78 270 bottom
C52  23.62,28.78 90 bottom
C53  72.26,32.72 0 bottom
C54  65.28,36.91 180 top
D1  84.29,43.17 180 top
D2  24.6,17.27 180 bottom
D3  14.99,30.05 180 bottom
D5  4.97,20.73 180 top
D6  18.59,45.48 0 top
D8  18.92,17.06 180 top
FID1  89.37,49.84 0 top
FID2  95,1.09 0 top
FID3  8.13,51.39 0 bottom
FID4  8.89,51.39 0 top
FID5  88.86,49.84 0 bottom
FID6  95,4.9 0 bottom
J1  9.56,13.08 0 top
J2  17.81,13.12 0 top
J3  69.09,47.58 0 top
J4  94.23,33.1 90 top
J5  76.96,7.44 90 top
J6  47.05,34.44 0 top
K1  16.76,22.43 270 bottom
L1  83.15,46.78 90 top
L2  28.87,41.98 90 top
L3  76.71,3 270 top
L4  79.76,7.14 270 top
L5  30.35,22.3 0 top
L6  29.97,27.89 0 top
L7  47.4,26.6 90 top
LED1  63.41,47.65 0 top
LED2  41.55,23.7 0 top
LED3  65.84,23.7 0 top
LK2  10.92,21.92 270 bottom
LK3  22.61,21.92 270 bottom
OP1  83.84,3.13 270 top
PTC1  11.98,19.24 270 top
Q1  45.92,23.4 180 top
Q2  64.08,43.26 0 top
Q3  9.65,24.97 180 top
Q9  81.67,29.47 180 bottom
R1  38.1,33.86 180 top
R2  74.3,35.77 0 top
R3  22.42,31.05 90 top
R4  24.19,31.05 90 top
R5  25.97,31.05 90 top
R6  27.75,31.05 90 top
R7  31.31,31.05 90 top
R8  29.53,31.05 90 top
R9  20.49,31.04 90 top
R10  18.63,31.04 90 top
R11  20.35,36.22 0 top
R12  34.42,30.67 270 top
R13  2.43,29.97 270 top
R14  44.7,45.04 90 top
R15  73.7,41.57 0 top
R16  76.16,41.9 90 top
R17  47.24,45.04 90 top
R18  59.36,37.78 180 top
R19  88.62,11.24 180 bottom
R20  73.53,25.35 180 top
R21  49.78,45.04 90 top
R22  78.99,4.52 180 bottom
R23  55.77,34.04 270 top
R24  52.32,45.04 90 top
R25  68.71,28.91 90 top
R26  79.03,2.19 180 bottom
R27  90.81,22.56 0 top
R28  81.93,32.01 0 bottom
R29  54.86,45.04 90 top
R30  79.76,23.45 180 top
R31  61.67,42.66 90 top
R32  78.69,33.45 180 top
R33  64.77,29.66 0 top
R35  59.65,42.72 90 top
R36  26.06,12.65 180 top
R37  26.06,16.21 0 top
R38  42.47,28.48 180 top
R39  66.12,34.25 270 top
R40  70.51,22.99 180 top
R43  8.97,35.87 90 bottom
R44  20.64,41.23 0 top
R52  76.2,17.1 90 top
R53  76.96,24.46 90 top
R54  90.93,6.94 180 top
R57  79.9,36.58 90 top
R58  87.01,32.26 0 bottom
R61  79.54,29.68 90 bottom
R65  15.32,34.25 180 top
R66  56.39,45.04 90 top
R77  78.12,36.58 90 top
R99  88.65,13.67 0 bottom
S1  86,15.32 180 top
S2  10.67,30.3 180 top
TP1  22.96,13.96 0 top
TP2  49.83,25.45 0 top
TP3  28.07,18.11 0 top
TP4  64.14,39.83 0 top
TP5  94.49,15.32 0 top
TP6  31.75,26.24 0 top
TP7  31.75,24.08 0 top
TP8  15.37,25.22 0 top
TP9  62.1,27.76 0 top
TP10  66.8,39.83 0 top
TP11  15.49,21.29 0 top
TP12  22.48,12.14 0 top
TP13  94.23,24.21 0 top
TP14  19.15,51.13 0 top
U1  85.99,30.23 0 top
U2  78.96,41.39 0 top
U3  73.03,30.43 0 top
U4  36.65,36.7 0 top
U5  55.88,26.75 270 top
U6  60.96,33.35 270 top
U7  23.05,24.96 180 top
U8  14.24,38.75 0 top
X1  78.75,28.01 90 top

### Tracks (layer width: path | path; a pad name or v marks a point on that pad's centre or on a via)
AREF  (via drill 0.3 pad 0.64)
  Top 0.305: U1.20 87.28,29.83 v87.12,29.67
  Bottom 0.305: v87.12,29.67 86.74,29.67 86.61,29.8 86.61,30.23 C32.2
BUZZ  (via drill 0.3 pad 0.64)
  Top 0.406: U1.10 83.99,29.71 84.33,30.05 v84.33,31.07
  Bottom 0.406: v84.33,31.07 84.33,31.32 83.64,32.01 R28.1
CHG_POL
  Top 0.406: R30.1 83.57,23.45 84.79,24.67 U1.11
CS
  Top 0.406: J6.7
  Top 0.61: J6.7 R29.2 R66.2
D0
  Top 0.406: J6.3
  Top 0.61: R14.2 J6.3
D1
  Top 0.406: J6.4
  Top 0.61: R17.2 J6.4
DSP_RST  (via drill 0.3 pad 0.64)
  Top 0.406: U1.12 85.59,26.75 85.09,27.26 85.09,29.41 85.72,30.05 85.72,32.72 85.09,33.35 v84.84,33.35 | R21.1 49.78,40.46 v52.58,37.67
  Bottom 0.406: v52.58,37.67 53.85,36.4 65.02,36.4 66.65,34.77 72.95,34.77 73.36,35.18 83.01,35.18 v84.84,33.35
DTR
  Top 0.406: C33.2 91.16,34.65 91.44,34.37 91.44,31.57 92.46,30.56 92.46,28.53 J4.P$1
EN_DCDC  (via drill 0.3 pad 0.64)
  Top 0.406: U8.3 10.22,38.11 v9.91,38.43 | R31.1 61.67,40.77 v61.72,40.72 | U1.24 89.38,33.03 v88.9,33.3
  Bottom 0.406: R43.2 8.97,38 9.4,38.43 v9.91,38.43 9.91,40.72 11.43,42.24 61.21,42.24 61.72,41.73 v61.72,40.72 61.67,40.77 R31.1 62.15,42.24 65.53,42.24 65.79,41.99 67.56,41.99 68.83,40.72 76.45,40.72 77.98,42.24 82.04,42.24 82.8,41.48 87.83,41.48 89.31,40.01 89.31,33.76 v88.9,33.3
GND  (via drill 0.3, 0.3 pad 0.64, 0.41 pad 0.81, 0.41 pad 0.91)
  Top 0.305: C21.2 1.08,33.03 v0.89,32.84 | 3.53,38 C17.2 | 6.64,36.18 v6.6,36.15 | 19.4,39.38 C38.1 19.43,39.36 | 14.87,39.38 U8.PAD | U1.3 82.57,31.43 v83.31,30.68 82.45,29.83 U1.5 | 85.98,43.21 D1.+ | 6.97,14.69 v6.99,14.68 | 35.38,38.74 v35.31,38.81 | 57.48,30.39 v57.4,30.3 58.03,30.93 U6.7 | 54.49,39.44 v54.48,39.45 | 78.58,41.39 v78.61,41.35 | 8.91,37.67 C28.1
  Top 0.406: 85.69,42.92 D1.+ | 86.61,45.47 C4.2 | X1.2 | C45.1 77.27,30.71 v76.83,31.14 76.96,31.27 76.96,31.73 77.79,32.55 R32.2 | U3.7 75.95,27.51 v77.09,26.37 | 44.59,24.32 v44.3,24.61
  Top 0.61: Q3.2 9,25.46 8.76,25.22 C35.2 6.99,26.74 v6.86,26.88 6.17,27.57 S2.2 | C2.1 2.03,24.72 v1.78,24.46 | C18.2 3.53,38 | C10.1 6.22,35.76 v6.6,36.15 | C18.2 6.64,36.18 | 19.4,39.38 U8.7 14.87,39.38 | 19.43,39.36 19.43,40.08 19.74,40.39 R44.1 19.74,42.77 v19.3,43.21 | D6.1 13.83,45.48 v13.64,45.29 | C34.1 24.07,36.39 v24.21,36.53 | U1.21 88.96,30.63 v88.9,30.68 | C4.2 87.97,45.5 v88.14,45.67 | C12.1 95.01,20.26 v95.12,20.14 | C24.1 95.01,8.83 v95.12,8.71 | TP1.1 23.51,14.43 C13.1 R36.2 24.26,12.65 v24,12.4 | D8.A 16.57,18.68 v16,19.26 | C36.1 6.97,14.69 | U7.10 U7.9 17.8,22.16 17.53,22.43 v17.53,23.06 | v18.54,26.37 18.61,26.43 U7.8 U7.7 | C44.1 27.97,24.11 v27.56,23.7 27.5,23.64 U7.16 | U4.2 U4.1 35.38,38.74 | C26.2 39.49,43.76 39.99,44.26 C25.1 39.99,47.78 J6.1 | C7.1 55.8,23.15 v56.01,22.94 | U5.3 57.92,26.75 v58.04,26.88 | C11.1 57.19,30.09 v57.4,30.3 | C49.1 67.58,33.11 67.31,32.84 v67.31,32.41 | C47.1 v72.26,37.29 | C54.1 v67.31,36.91 | C9.2 54.49,39.44 | R16.2 75.14,42.8 v75.06,42.88 | U2.2 78.58,41.39 | X1.2 79.74,28 v80.14,27.64 | C46.1 89.52,24.32 v89.28,24.08 | C18.2 7.8,38 8.13,37.67 8.91,37.67 | Q2.2 66.46,42.33 v67.06,43 | R18.1 60.26,34.56 v59.94,34.24 | C6.2 85.69,42.92 | 85.98,43.21 85.98,44.15 86.61,44.78 86.61,45.47 | C8.1 51.75,25.59 v51.74,25.58 | OP1.3 85.83,1.86 v85.7,1.73 | C14.1 64.44,26.5 v64.36,26.42 | C48.1 75.21,23.01 v75.44,22.79 | Q1.2 44.59,24.32
  Bottom 0.305: C30.1 10.85,34.97 R43.1 8.97,34.09 v9.14,33.91 | C42.2 C40.2 C39.2 | 34.67,37.71 C41.2 34.67,37.81 | 88.85,30.74 v88.9,30.68 | Q9.2 83.02,30.39 v83.31,30.68 | 23.36,29.92 C52.2
  Bottom 0.406: K1.2 20.26,23.25 | 88.13,45.66 v88.14,45.67 | C27.1 77.16,31.47 v76.83,31.14 | C1.1 95.03,42.54 v94.56,43 | 81.84,15.64 C23.1
  Bottom 0.61: 34.67,37.71 C39.2 31.71,38.6 v31.5,38.81 | K1.5 15.38,18.63 v16,19.26 | v35.31,38.81 34.92,38.81 34.67,38.56 34.67,37.81 | C50.1 v73.41,44.53 | LK3.1 22.61,23.06 v23.5,23.95 | C53.1 73.76,32.72 v74.3,32.18 | C31.1 85.88,27.74 v85.98,27.64 | C32.1 88.85,30.74 | 23.36,29.92 22.61,29.92 22.36,29.68 C51.1 21.59,30.56 19.94,32.21 v19.94,32.97 | C22.1 82.92,12.39 v83.06,12.52 | C23.1 80.76,15.69 v80.64,15.57 | D2.1 23.65,19.92 v23.62,19.89 | 20.26,23.25 19.81,23.7 v18.67,23.7 | C20.1 60.72,33.47 v59.94,34.24 | C15.1 88.13,45.66 | R22.2 82.73,4.52 v83.06,4.19 | C16.1 81.84,15.64
  other vias: 15.11,39.96 14.35,39.96 13.59,39.96 13.34,39.19 14.1,39.19 14.86,39.19 15.11,38.43 14.35,38.43 13.59,38.43 13.34,37.67 14.1,37.67 14.86,37.67
  pour GND (isolate 0.305): 0,11 0,44.91 0,45.04 8,53.04 87.88,53.04 96.01,44.91 96.01,-0.05 74.8,-0.05 74.8,21.03 29.34,21.03 29.34,11
  pour Bottom: 12.04,41.58 12.04,37.52 12.9,36.65 12.9,35.38 13.67,34.62 15.95,34.62 17.58,36.25 18.44,37.11 18.44,40.16 18.64,40.36 18.85,40.57 18.85,41.28 18.54,41.58
ISENSE  (via drill 0.3 pad 0.64, 0.41 pad 0.91)
  Top 0.406: U6.13 63.38,34.65 63.09,34.37 62.79,34.37 62.48,34.67 62.48,36.15 63.5,37.16 63.5,39.19 TP4.1 65.38,38.58 67.72,38.58 68.58,39.45 v68.58,42.24 | U4.3 33.91,35.77 v33.78,35.89 | U1.22 89.05,31.43 v88.9,31.57
  Bottom 0.406: v33.78,35.89 36.32,35.89 36.83,36.4 36.83,40.46 37.85,41.48 54.86,41.48 57.4,39.04 63.5,39.04 TP4.1 | v88.9,31.57 89.56,31.57 90.02,32.18 90.02,40.11 87.88,42.24 83.06,42.24 82.3,43 77.72,43 76.2,41.48 69.34,41.48 v68.58,42.24
MISO  (via drill 0.3 pad 0.64, 0.41 pad 0.91)
  Top 0.406: R24.1 53.22,44.14 v53.59,43.77 | U1.16 88.79,26.86 v88.14,27.51
  Top 0.61: v68.07,43.77 68.07,46.56 J3.1
  Bottom 0.406: v53.59,43.77 65.28,43.77 J3.1 | v88.14,27.51 88.14,27.76 88.65,28.27 90.42,28.27 90.93,28.78 90.93,32.08 90.63,32.49 90.63,40.36 87.73,43.26 83.06,43.26 82.3,44.02 74.42,44.02 72.64,42.24 69.6,42.24 v68.07,43.77
MOSI  (via drill 0.3 pad 0.64)
  Top 0.406: R17.1 48.4,44.14 v48.51,44.02 | U1.15 87.99,24.86 v88.14,24.72
  Bottom 0.406: v48.51,44.02 48.77,43.77 52.07,43.77 52.83,44.53 64.77,44.53 67.31,47.07 67.31,50.62 68.33,51.64 70.87,51.64 71.63,50.88 | 71.63,50.88 J3.4 | v88.14,24.72 88.14,24.97 89.92,26.75 91.03,26.75 92.46,28.17 92.46,32.59 91.95,33.1 91.95,40.97 88.14,44.78 83.82,44.78 76.96,51.64 72.39,51.64 71.63,50.88
N$1
  Top 0.406: U7.6 21.14,29.1 22.2,30.15 R3.1 22.35,30.09
N$2
  Top 0.406: U7.5 22.42,28.59 23.92,30.09 24.13,30.09 R4.1
N$3
  Top 0.406: U7.4 23.69,28.59 24.13,29.03 24.6,29.03 25.72,30.15 R5.1
N$4
  Top 0.406: U7.3 24.96,28.34 25.65,29.03 26.63,29.03 R6.1
N$5  (via drill 0.3 pad 0.64)
  Top 0.406: R7.1 31.3,29.48 v31.5,29.29 | U7.14 24.96,21.1 25.65,20.4 27.18,20.4 v27.43,20.14
  Bottom 0.406: v31.5,29.29 29.72,27.51 29.72,23.19 27.43,20.91 v27.43,20.14
N$6
  Top 0.406: J6.6
  Top 0.61: R24.2 J6.6
N$7  (via drill 0.3 pad 0.64)
  Top 0.406: R8.1 29.53,29.61 v29.21,29.29 | U7.13 23.69,21.1 25.15,19.64 v26.67,19.64
  Bottom 0.406: v29.21,29.29 29.21,28.53 28.96,28.27 28.96,23.45 26.67,21.16 v26.67,19.64
N$8
  Top 0.406: U7.12 22.42,24.4 21.34,25.48 18.03,25.48 17.53,25.99 17.53,28.53 18.03,29.03 20.07,29.03 20.48,29.45 R9.1
N$9
  Top 0.406: U7.11 21.14,24.4 20.83,24.72 17.78,24.72 16,26.49 13.46,26.49 12.7,27.26 12.7,29.29 13.46,30.05 18.54,30.05 R10.1
N$10
  Top 0.406: U4.4 38.73,35.77 | R1.1 39,35.5 38.73,35.77 | C43.2 40.02,37.05 38.73,35.77
N$11
  Top 0.61: R35.2 59.65,44.49 60.2,45.04 61.47,45.04 61.98,45.54 61.98,47.49 LED1.A
N$12
  Top 0.61: Q2.3 64.08,47.05 LED1.K
N$13
  Top 0.406: U6.6 58.7,32.05 59.18,31.57 59.18,28.78 61.47,26.49 62.99,26.49 63.46,26.97 63.46,29.25 R33.1
N$14
  Top 1.016: PTC1.1 10.03,21.84 8.94,20.75 8.09,20.75 D5.1
N$15
  Top 0.406: U6.12 64.96,34 65.33,34.37 65.79,34.37 66.12,34.7 R39.1
N$16
  Top 0.406: C3.1 78.06,43.08 77.68,42.71 U2.1
N$17
  Top 0.406: 6.1,32.23 S2.4 6.35,32.49
  Top 0.61: R13.1 5.65,30.87 6.1,31.32 6.1,32.23 | C10.2 5.99,33.96 6.35,33.61 6.35,32.49 | S2.4 10.64,32.3 12.59,34.25 R65.2
N$18
  Top 0.406: U3.9 74.33,35.29 74.8,35.77 R2.2 C47.2
N$19
  Top 0.406: C3.2 79.86,43.16 80.23,42.78 U2.6 81.12,42.34 81.95,43.17 D1.- 82.64,44.11 83.15,44.62 L1.1
N$20  (via drill 0.3 pad 0.61)
  Top 0.406: v78.94,32.28 78.94,32.81 R32.1
  Bottom 0.305: v78.94,32.28 78.94,32.39 79.3,32.74 80.26,32.74 80.37,32.64 80.39,32.64 R28.2
  Bottom 0.406: Q9.1 R28.2
N$21
  Top 0.61: R31.2 62.69,43.56 63.43,42.82 Q2.1
N$22
  Top 0.406: U3.10 73.67,34.86 73.41,35.13 73.41,35.75 R2.1
N$23
  Top 0.406: U3.6 74.33,25.46 R20.1
N$24
  Top 0.406: X1.1 81.08,26.8 U1.8
N$25
  Top 0.406: U3.2 71.72,28.33 71.37,28.68 70.1,28.68 69.44,28.02 R25.1
N$26
  Top 0.406: R25.2 C49.2 71.37,31.32 71.72,31.67 U3.13
N$27
  Top 0.406: R15.2 C5.1 75.78,39.79 76.16,40.17 | R16.1 76.16,40.17 | U2.3 77.68,39.91 77.47,39.7 76.63,39.7 76.16,40.17
N$28
  Top 0.406: U3.3 72.38,26.26 72.64,25.99 72.64,25.36 R20.2 72.68,25.3 C48.2
N$29
  Top 0.406: C11.2 R23.2 55.77,33.75 56.02,34 U6.3
N$30
  Top 0.406: R27.1 89.43,22.56 87.99,24.01 87.58,24.01 86.39,25.19 U1.13
N$31  (via drill 0.41 pad 0.91)
  Top 0.406: OP1.4 87.57,5.91 v88.7,7.04
  Bottom 0.406: R19.1 87.72,10.86 87.73,10.85 87.73,10.54 88.7,9.58 v88.7,7.04
  Bottom 0.61: TP5.1 92.25,15.32 90.6,13.67 R99.1 87.72,11.84 R19.1
N$32  (via drill 0.3 pad 0.64)
  Top 0.406: L7.2 47.4,29.61 BZ1.1 47.14,31.52 v47.55,31.93
  Bottom 0.406: 79.24,30.28 R61.2 79.55,30.57 79.55,29.95 79.28,29.67 C27.2 77.76,29.49 75.39,29.49 73.3,31.57 58.67,31.57 58.22,32.03 47.65,32.03 v47.55,31.93
N$33
  Top 0.406: PTC1.2
  Top 0.813: C36.2 8.77,16.22 9.14,16.59 PTC1.2 | PTC1.2 11.98,13.34 J1.2
N$34
  Top 0.406: U6.2 56.81,34.65 56.59,34.88 55.83,34.88 R23.1
N$36
  Top 0.406: U1.7 80.82,28.23 79.84,29.2 X1.3
N$37
  Top 0.406: U6.9 64.7,32.05 65.23,31.52 65.23,30.91 65.63,30.51 65.63,29.69 R33.2 65.67,29.05 66.04,28.68 66.04,28.09 C14.2
N$38
  Top 0.61: LED2.A 40.28,25.07 41.57,26.36 R38.2
N$39
  Top 0.406: R39.2 66.55,33.35 67.31,34.11 67.31,35.38 68.33,36.4 68.33,37.42 67.82,37.92 64.77,37.92 64.38,37.53 C54.2 | U6.11 R39.2 | R39.2
N$40  (via drill 0.3 pad 0.64)
  Top 0.406: U7.2 26.23,26.68 v26.42,26.49 | L6.1 29.07,28.16 v28.19,29.03
  Bottom 0.406: v28.19,29.03 26.42,29.03 25.91,28.53 25.91,27 v26.42,26.49
N$41  (via drill 0.41 pad 0.91)
  Top 0.406: OP1.2 82.09,1.86 v82.35,2.11
  Bottom 0.406: v82.35,2.11 80.71,2.11 R26.2
N$42  (via drill 0.3 pad 0.64, 0.41 pad 0.91)
  Top 0.406: v68.48,22.68 67.31,21.52 39.06,21.52 38.2,22.38 38.2,24.82 40.44,27.05 40.44,29.49 v40.39,29.54 | R30.2 78.86,24.58 v79.35,25.07
  Top 0.61: Q3.1 11.34,25.89 v11.43,25.99
  PWR 0.406: v68.48,22.68 68.68,22.89 68.68,23.8 69.14,24.26 78.54,24.26 v79.35,25.07
  Bottom 0.406: v11.43,25.99 11.43,31.32 13.72,33.61 19.05,33.61 19.3,33.86 20.32,33.86 22.3,31.88 31.95,31.88 33.78,30.05 39.88,30.05 v40.39,29.54
N$43  (via drill 0.41 pad 0.91)
  Top 0.406: L3.2 75.45,2.1 v75.54,2.11
  Bottom 0.406: v75.54,2.11 77.76,2.11 R26.1
N$44  (via drill 0.3 pad 0.64)
  Top 0.406: U8.4 11.36,36.47 v11.94,35.89
  Bottom 0.406: v11.94,35.89 11.9,35.89 C30.2
N$46  (via drill 0.3 pad 0.64)
  Top 0.406: v76.2,5.67 76.57,6.04 78.55,6.04 78.75,6.24 L4.2
  Bottom 0.406: v76.2,5.67 76.2,4.9 76.58,4.52 R22.1
N$47
  Top 0.406: 11.23,40.78 U8.1
  Top 0.61: C29.1 11.23,40.78
N$48
  Top 0.406: 19.45,34.7 C19.1 19.37,34.62 18.8,34.62 18.63,34.46 R10.2 R9.2 22.4,31.94 R3.2 R4.2 R5.2 R6.2 R8.2 R7.2 | R11.1 17.45,36.22 17.11,36.56 U8.5
  Top 0.61: R11.1 19.45,34.7
N$49
  Top 0.61: R40.2 69.61,24.09 68.28,25.43 66.29,25.43 LED3.A
N$51
  Top 0.406: U8.8 17.11,41.13 16.76,41.48
  Top 0.61: C29.2 13.03,41.91 13.46,41.48 16.76,41.48 17.78,42.5 17.78,44.53 18.73,45.48 D6.2
  Top 1.016: D6.2 23.69,45.48 28.87,40.3 L2.1
N$52
  Top 0.406: 19.51,37.48 C38.2
  Top 0.61: C37.2 19.51,37.48 | U8.6 18.87,38.11 C38.2
N$53
  Top 0.61: R44.2 21.54,39.34 C37.1
N$54
  Top 0.406: U7.15 26.23,21.35 26.54,21.03 28.07,21.03 28.45,21.41 28.45,21.92 28.83,22.3 L5.1
N$55
  Top 0.406: L3.1 75.88,3.9 75.44,4.34 75.44,6.68 75.95,7.19 76.83,7.19 J5.1
N$56
  Top 0.406: L4.1 79.76,9.27 78.92,10.11 J5.2
N$57
  Top 0.406: Q1.3 44.05,22.47 LED2.K
  Bottom 0.406: LED3.K 67.11,22.02 66.55,21.46 45.06,21.46 LED2.K
N$64  (via drill 0.3 pad 0.64)
  Top 0.406: v50.6,31.12 50.19,31.12 49.17,32.13 49.17,34.57 47.14,36.6 BZ1.2
  Bottom 0.406: Q9.3 80.76,28.54 80.52,28.78 R61.1 75.08,28.78 73.05,30.81 58.42,30.81 57.91,31.32 50.8,31.32 v50.6,31.12
OVC_ALARM  (via drill 0.3 pad 0.64, 0.41 pad 0.81)
  Top 0.406: TP10.1 65.41,41.23 63.5,41.23 62.79,40.52 62.79,37.36 61.82,36.4 61.82,33.71 62.83,32.7 U6.10 65.06,32.7 67.26,30.51 67.26,27.46 v67.46,27.05 | v80.97,25.12 81.69,25.83 83.09,25.83 U1.9
  Bottom 0.406: v80.97,25.12 80.06,24.21 78.03,24.21 75.79,26.44 71.32,26.44 70.92,26.85 67.67,26.85 v67.46,27.05
PEDAL_IP  (via drill 0.3 pad 0.64)
  Top 0.406: U6.4 59.94,33.35 v60.96,32.34 | U1.32 82.65,34.52 v82.5,34.37
  Bottom 0.406: v82.5,34.37 73.56,34.37 73.15,33.96 65.23,33.96 63.8,32.54 61.16,32.54 v60.96,32.34
PUSH  (via drill 0.3 pad 0.64)
  Top 0.406: TP9.1 60.2,29.67 60.2,31.83 v59.44,32.59 59.32,32.7 U6.5 | R65.1 17.16,34.25 v17.27,34.37
  Bottom 0.406: v59.44,32.59 59.32,32.7 56.47,32.7 51.76,37.42 46.23,37.42 39.62,30.81 34.04,30.81 32.21,32.64 22.81,32.64 20.83,34.62 17.53,34.62 v17.27,34.37
PUSH_FILT  (via drill 0.3 pad 0.64)
  Top 0.406: U1.25 88.79,37.12 v88.44,37.47 | U6.8 62.3,31.4 61.77,31.93 61.77,32.74 61.21,33.3 61.21,37.16 61.98,37.92 v61.98,39.8
  Bottom 0.406: v61.98,39.8 63.4,41.23 67.31,41.23 68.58,39.96 82.91,39.96 83.67,40.72 87.68,40.72 88.65,39.75 88.65,37.67 v88.44,37.47
RESET
  Top 0.406: 75.69,38.43 70.61,38.43 69.34,39.7 69.34,44.02 70.87,45.54 73.41,45.54 74.17,46.31 J3.5 | 75.69,38.43 76.2,38.94 79.76,38.94 80.26,39.45 83.82,39.45 85.6,37.67 | C33.1 90.39,36.95 88.9,38.43 86.36,38.43 85.6,37.67 | U1.29 85.6,37.67 | R77.1 76.67,35.68 76.2,36.15 76.2,36.81 76.1,36.91 76.1,38.03 75.69,38.43
ROTA
  Top 0.406: 78.49,17.88 S1.A | U3.5 73.67,26.13 73.53,25.99 73.53,24.59 73.79,24.34 75.06,24.34 75.82,23.57 76.95,23.57 R53.1
  Top 0.61: R53.1 76.96,19.99 78.49,18.47 78.49,17.88
  Bottom 0.61: C23.2 78.88,17.49 S1.A
ROTA_FILT  (via drill 0.3 pad 0.64)
  Top 0.406: U1.2 83.46,32.23 v84.07,32.84 | U3.4 73.03,28.09 75.69,30.76 v75.69,32.59
  Bottom 0.406: v84.07,32.84 84.07,33.1 83.82,33.35 76.45,33.35 v75.69,32.59
ROTB  (via drill 0.3 pad 0.64)
  Top 0.406: S1.B | U3.11 73.03,29.36
  Top 0.61: R52.1 76.2,14.05 77.47,12.78 S1.B | v85.85,14.05 79.78,14.05 S1.B | 73.03,29.36 v72.49,28.83
  Bottom 0.61: C22.2 79.91,14.19 S1.B | v85.85,14.05 85.6,14.3 85.6,18.67 83.26,21.01 83.26,24.66 81.94,25.99 79.5,25.99 78.23,27.26 74.57,27.26 73,28.83 v72.49,28.83
ROTB_FILT
  Top 0.406: U1.1 81.7,33.7 80.77,34.62 75.44,34.62 74.98,34.16 U3.8
ROTPUSH  (via drill 0.3 pad 0.64)
  Top 0.406: U3.1 71.08,26.04
  Top 0.61: R54.1 91.83,9.87 92.59,10.63 C24.2 93.98,11.79 S1.SW+ 92.98,15.55 90.02,18.52 v81.89,18.52 | 71.08,26.04 v70.05,25.02
  Bottom 0.61: v70.05,25.02 70.61,24.46 75.13,24.46 81.08,18.52 v81.89,18.52
RPUSH_FILT  (via drill 0.3 pad 0.64)
  Top 0.406: U3.12 72.38,35.77 v71.98,36.2 | U1.26 87.99,35.58 87.68,35.89 v87.25,35.89
  Bottom 0.406: v87.25,35.89 87.25,35.26 86.87,34.88 85.85,34.88 84.33,36.4 72.19,36.4 v71.98,36.2
RST
  Top 0.406: J6.5
  Top 0.61: R21.2 J6.5
RX-I  (via drill 0.3 pad 0.64)
  Top 0.406: J4.P$3 93.47,31.83 92.84,32.46 92.84,37.03 89.92,39.96 87.38,39.96 v86.61,39.19 | v83.82,38.43 84.79,37.46 U1.30
  Bottom 0.406: v86.61,39.19 84.58,39.19 v83.82,38.43
SCK  (via drill 0.3 pad 0.64)
  Top 0.406: R14.1 44.7,43.51 v45.21,43 | U1.17 89.24,27.43 v89.15,27.51
  Bottom 0.406: v45.21,43 65.79,43 68.33,45.54 69.85,45.54 J3.3 73.41,45.54 82.04,45.54 83.57,44.02 87.88,44.02 91.29,40.62 91.29,32.74 91.69,32.34 91.69,28.42 90.78,27.51 v89.15,27.51
SCL  (via drill 0.3 pad 0.64)
  Top 0.406: L5.2 31.25,23.58 TP7.1 | 79.94,35.64 R57.1 80.96,35.68 81.48,36.2 v81.48,37.16 | U1.28 86.39,35.86 v86.36,35.89 | v39.37,31.83 39.37,27.51 v38.86,27
  Bottom 0.406: TP7.1 31.75,24.46 34.29,27 v38.86,27 | v39.37,31.83 45.97,38.43 55.63,38.43 56.24,37.82 68.28,37.82 69.09,38.64 80.06,38.64 81.48,37.21 v81.48,37.16 81.74,37.01 85.75,37.01 86.36,36.4 v86.36,35.89
SDA  (via drill 0.3 pad 0.64)
  Top 0.406: U1.27 87.19,33.42 v87.12,33.35 | L6.2 31.37,27.89 31.75,27.51 TP6.1 | v38.35,32.08 38.35,28.27 v37.85,27.76
  Bottom 0.406: R58.1 87.45,32.26 87.12,32.59 v87.12,33.35 87.68,33.35 88.09,33.76 88.09,36.2 86.67,37.62 82.3,37.62 80.67,39.25 68.68,39.25 67.87,38.43 56.9,38.43 54.61,40.72 46.99,40.72 v38.35,32.08 | TP6.1 32.51,26.24 34.04,27.76 v37.85,27.76
SPARE  (via drill 0.3 pad 0.64, 0.41 pad 0.81, 0.41 pad 0.91)
  Top 0.305: U6.1 58.03,36.07 57.51,36.6 56.09,36.6 C9.1
  Top 0.406: 56.07,36.65 C9.1 56.06,37.34 56.5,37.78 R18.2 | U6.1 58.96,35.3 v59.08,35.18 | U1.23 89.31,32.23 v88.9,32.44
  PWR 0.406: v86.87,15.95 86.87,16.84 81.79,21.92 81.79,35 84.58,37.8 | 84.58,37.8 84.58,40.97 83.44,42.11 73.15,42.11 69.6,38.56 69.57,38.56 68.94,37.92 64.01,37.92 61.21,35.13 59.13,35.13 v59.08,35.18 | v88.9,32.44 88.29,32.44 87.99,32.74 87.99,36.2 87.38,36.81 85.57,36.81 84.58,37.8
  Bottom 0.61: v86.87,15.95 86.87,14.54 R99.2
SS  (via drill 0.3 pad 0.64)
  Top 0.406: R29.1 54.86,41.73 53.59,40.46 53.59,37.92 v53.85,37.67 | U1.14 87.19,27.95 86.36,28.78 86.36,33.1 v86.11,33.35
  Bottom 0.406: v53.85,37.67 54.51,37.01 65.43,37.01 67.06,35.38 72.54,35.38 72.95,35.79 83.72,35.79 86.11,33.4 v86.11,33.35
TEST  (via drill 0.3 pad 0.25, 0.3 pad 0.64)
  Top 0.406: TP13.1 92.2,24.21 91.7,23.71 R27.2 91.7,20.61 90.42,19.33 79.05,19.33 v78.64,19.74 | Q1.1 46.57,23.76 47.14,23.19 v49.78,23.19
  Bottom 0.406: v49.78,23.19 50.6,23.19 51.61,24.21 55.68,24.21 57.51,26.04 63.2,26.04 64.01,25.22 68.07,25.22 69.7,23.6 73.36,23.6 75.18,21.77 76.61,21.77 v78.64,19.74
TX-O  (via drill 0.3 pad 0.64)
  Top 0.406: J4.P$2 94.23,29.8 92.08,31.95 92.08,36.78 89.66,39.19 v87.88,39.19 | U1.31 83.99,37.04 82.8,38.23 v82.8,38.43
  Bottom 0.406: v87.88,39.19 87.88,39.45 87.38,39.96 83.97,39.96 82.8,38.79 v82.8,38.43
VCC  (via drill 0.41 pad 0.91, 0.89 pad 1.68)
  Top 0.305: 3.53,41.2 C17.1 3.46,41.23 | 8.99,39.38 C28.2 | 82.8,40.97 C6.1
  Top 0.61: C18.1 3.53,41.2 | C18.1 6.64,42.33 v6.48,42.5 | U8.2 8.99,39.38 | C6.1 82.64,40.93 81.7,40.93 v81.53,41.1 80.88,40.44 U2.4 U2.5 | C21.1 1.18,36.23 0.76,36.65 0.76,40.72 1.27,41.23 3.46,41.23 | U5.2 56.06,25.8 v55.98,25.68 | C28.2 8.43,39.41 C18.1 | C7.2 53.12,23.06 v52.07,23.06 | L7.1 47.4,24.97 v47.75,24.61
  Top 1.016: v4.45,18.54 4.45,19.97 3.66,20.75 3.45,20.75 | 3.45,20.75 1.89,20.75 D5.2 | C35.1 4.19,21.49 3.45,20.75
  pour PWR (isolate 0.305): 4.45,43.38 10.92,43.38 10.92,24.97 31.24,25.1 31.24,26.62 61.09,26.75 61.09,28.4 71.63,28.4 71.63,39.7 73.41,41.48 83.31,41.48 83.31,38.94 76.2,38.94 74.93,37.67 74.93,24.84 68.2,24.72 64.9,21.03 29.34,20.91 29.34,11 0,11 0,26.49 4.45,26.49
VCC-ISO  (via drill 0.41 pad 0.81, 0.41 pad 0.91)
  Top 0.305: 41.78,45.3 C25.2 | C26.1 | 2.41,29.06 R13.2 | 83.24,48.08 L1.2 | 58.42,40.72 v58.42,40.97 | 1.06,29.07 v1.02,29.03 | 27.76,25.91 v27.69,25.99
  Top 0.406: U6.14 63.58,35.3 v63.37,35.51 | U1.4 79.64,30.63 C45.2 79.64,31.51 v79.91,31.78
  Top 0.508: U3.14 70.62,33.36 v70.23,32.97
  Top 0.61: J6.2 42.17,46.95 41.78,46.56 41.78,45.3 | C25.2 41.79,44.26 42.29,43.77 C26.1 | U1.6 83.06,29.03 v83.19,28.91 | C2.2 2.03,28.02 2.41,28.4 2.41,29.06 | R54.2 90.03,8.09 v89.92,8.21 | C12.2 95.13,22.06 v95.25,22.18 | C46.2 91.32,26.12 v91.69,25.99 91.69,28.02 91.48,28.23 U1.18 | R52.2 v76.2,18.87 | R53.2 78.09,25.36 v78.23,25.22 | R57.2 R77.2 77.02,37.48 v76.96,37.42 | C4.1 85.56,48.3 85.34,48.08 83.24,48.08 | L1.2 83.15,49.77 v82.8,50.12 | C5.2 R15.1 72.8,42.85 72.39,43.26 v70.61,43.26 | R35.1 58.77,41.83 58.42,41.48 v58.42,40.97 | R66.1 v56.39,41.23 | R13.2 1.06,29.07 | C44.2 27.76,25.91 | U7.1 27.5,26.18 v27.69,25.99 | R40.1 71.41,22.09 v71.73,21.77 | R38.1 44.09,28.48 v44.3,28.68
  Bottom 0.305: 84.03,28.91 C31.2 | 62.24,35.26 C20.2 | v21.83,26.23 v21.84,26.24
  Bottom 0.406: 62.24,35.26 63.12,35.26 v63.37,35.51 | J4.P$4 93.73,34.37 92.71,35.38 92.71,41.16 C1.2
  Bottom 0.61: v83.19,28.91 84.03,28.91 | C15.2 86.61,49.86 v86.36,50.12 | C50.2 70.73,43.37 v70.61,43.26 | D3.2 17.19,31.15 v17.27,31.07 | C52.1 v23.62,25.99 | K1.1 v21.83,26.23 | C51.2 21.59,26.49 v21.84,26.24 | v27.69,25.99 25.55,23.85 D2.2 | R58.2 85.17,32.26 v84.84,32.08 | C53.2 70.48,32.72 v70.23,32.97 | R19.2 89.52,8.6 v89.92,8.21
  pour PWR (isolate 0.305, rank 2): 0,26.75 0,45.04 7.87,52.91 88.14,52.91 96.01,45.04 96.01,0.08 74.8,0.08 74.8,20.91 65.53,20.91 65.53,24.06 74.93,24.06 74.93,36.91 76.71,38.69 83.82,38.69 83.82,41.99 73.41,41.99 71.12,39.7 71.12,28.91 60.58,28.91 60.58,27.89 30.35,27.64 30.35,25.22 11.18,25.48 11.18,43.77 4.06,43.77 4.06,26.75
VCCIO  (via drill 0.41 pad 0.81)
  Top 0.61: TP2.1 49.84,26.16 51.06,27.39 C8.2 54.57,27.39 U5.1 55.87,27.7 v56.54,28.37 | OP1.1 81.38,4.4 81.79,4.8 v81.79,6.43
  Bottom 0.61: v81.79,6.43 81.79,8.66 84.73,11.61 84.73,17.81 | 84.73,17.81 84.73,18.26 82.8,20.2 80.77,20.2 75.54,25.43 71.12,25.43 70.51,26.04 66.85,26.04 63.6,29.29 60.55,29.29 59.74,28.48 56.64,28.48 v56.54,28.37 | C16.2 84.36,17.44 84.73,17.81
VO+
  Bottom 0.406: 13.21,20.89 K1.6
  Bottom 0.61: 13.21,20.89 13.21,21.41 13.11,21.51 LK2.2 10.92,20.4 11.43,19.89 11.43,16.84 15.15,13.12 J2.1 | K1.6 15.04,20.83 TP11.1
VO-
  Top 0.61: TP12.1 21.45,12.14 J2.2
  Bottom 0.61: LK3.2 22.61,21.16 22.28,20.83 | K1.3 22.28,20.83 | J2.2 20.47,15.22 22.61,17.35 22.61,20.5 22.28,20.83
VO_TPS  (via drill 0.41 pad 0.81, 0.41 pad 0.91)
  Top 0.406: U4.5 37.92,37.85 | R12.1 34.42,31.95 v34.54,31.83 | 21.25,34.7 C19.2 | 22.85,34.67 C34.2
  Top 0.61: R11.2 21.25,34.7 | C19.2 22.85,34.67
  Top 0.813: C43.1 37.22,38.55 37.92,37.85 | C34.2 22.94,33.78 v23.11,33.61 | v38.1,36.91 38.1,37.47 U4.5
  Top 1.016: L2.2 31.84,46.73 37.22,41.34 C43.1
  Bottom 0.406: C41.1 34.67,34.51 34.67,31.95 v34.54,31.83
  Bottom 0.813: 34.67,34.51 C39.1 C40.1 C42.1 25.74,33.95 25.4,33.61 v23.11,33.61 | C41.1 37.27,34.56 37.85,35.13 37.85,36.65 v38.1,36.91
  other vias: 26.47,49.86 27.33,49.86 28.19,49.86 29.06,49.86 29.92,49.86 31.5,49.3 30.78,49.81 31.6,48.39 31.85,47.42 31.8,46.61 31.75,45.75 31.7,44.88 31.19,44.17 30.33,43.87 30.99,43.41 31.95,43.77 32.46,44.53 32.51,45.44 32.61,46.31 32.41,48.13 31.65,50.22 30.43,50.57 29.46,50.67 28.45,50.73 27.53,50.73 26.62,50.73 26.11,48.95 26.06,48.13 26.01,47.32 25.96,46.46 25.91,45.65 27.94,43.66 28.75,43.66 29.57,43.66 32.66,47.27 25.35,48.64 25.3,47.78 25.25,46.97 25.25,46.2 25.45,49.76 25.7,50.62 12.45,51.54 13.31,51.54 9.6,48.69 9.6,47.73 9.55,46.66 10.52,46.56 10.31,49.51 11.18,50.42 14.63,51.59 15.8,51.64 17.07,51.69 20.83,51.59 21.64,51.64 22.61,51.69 23.57,51.69 11.63,47.07 12.45,47.68 11.79,50.98 24.49,51.69 25.1,51.18 26.06,51.64 27.43,51.74 28.91,51.74 30.38,51.59 32.51,49.2 24.74,50.37 24.69,49.35
  pour Top (isolate 0.813): 11.23,52.2 30.23,52.2 33.58,48.85 33.58,40.06 32.46,38.94 31.45,38.94 31.45,39.45 22.4,48.49 13.82,48.49 11.23,45.9 8.84,45.9 8.79,45.95 8.74,45.95 8.33,46.36 8.33,49 8.64,49.3 9.35,49.3 11.07,51.03 11.07,51.94 11.23,52.1
  pour Bottom (isolate 0.813): 12.4,52.2 8.84,48.64 8.84,44.83 10.57,43.11 32.11,43.11 33.38,44.38 33.78,44.38 33.99,44.58 33.99,50.62 32.41,52.2
VOSEN  (via drill 0.3 pad 0.64)
  Top 0.406: U1.19 88.13,29.03 v87.63,28.53
  Top 0.61: R36.1 C13.2 R37.2 26.96,17.64 27.43,18.11 TP3.1
  Bottom 0.406: 27.43,18.11 TP3.1 28.07,19 28.45,19.38 28.45,20.91 29.46,21.92 32.51,21.92 33.27,22.68 33.27,24.97 34.54,26.24 47.75,26.24 50.8,29.29 59.44,29.29 60.2,30.05 72.8,30.05 74.83,28.02 78.49,28.02 79.76,26.75 86.36,26.75 87.12,27.51 87.12,28.02 v87.63,28.53
  Bottom 0.61: D2.3 26.13,16.17 TP3.1
VOUT  (via drill 0.41 pad 0.91)
  Top 0.406: R12.2 34.42,28.14
  Top 0.61: R37.1 24,16.21 23.15,17.06 D8.C 21.27,19.06 v21.59,19.38 | R1.2 37.2,28.64 36.43,27.87 R12.2 | 34.42,28.14 v33.27,29.29
  Bottom 0.406: 20.32,18.69 K1.4 | 13.21,22.97 K1.7
  Bottom 0.61: v21.59,19.38 20.57,19.38 20.32,19.13 | 20.32,19.13 20.32,18.69 | LK2.1 13.1,22.32 13.21,22.43 13.21,22.97 | 20.32,19.13 20.07,19.38 17.53,19.38 16.89,20.02 16.89,22.05 15.91,23.03 | K1.7 15.91,23.03 | v33.27,29.29 32.26,30.3 26.67,30.3 25.15,28.78 25.15,25.73 24.38,24.97 17.85,24.97 15.91,23.03
VRELAY  (via drill 0.41 pad 0.91)
  Top 0.61: Q3.3 12.54,24.05 v13.21,24.72
  Bottom 0.406: v13.21,24.72 13.21,26.17 K1.8 | K1.8 13.26,28.33 13.89,28.95 D3.3 | K1.8 14.36,26.23 TP8.1

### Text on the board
tPlace: + | +5V | GND | RST | GND | + | + | +
bPlace: r8v0-DIC15 | V_TPS | #SER: | ISEN | OVC_ALARM | VRELAY | PUSH | 12V | SDA | SCL | TEST | VO+ | VO- | GND | OPTO_OP | VOSEN

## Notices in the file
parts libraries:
SparkFun-Electromechanical: Licensing: Creative Commons ShareAlike 4.0 International - https://creativecommons.org/licenses/by-sa/4.0
SparkFun-DiscreteSemi: Licensing: CC v3.0 Share-Alike You are welcome to use this library for commercial purposes.
